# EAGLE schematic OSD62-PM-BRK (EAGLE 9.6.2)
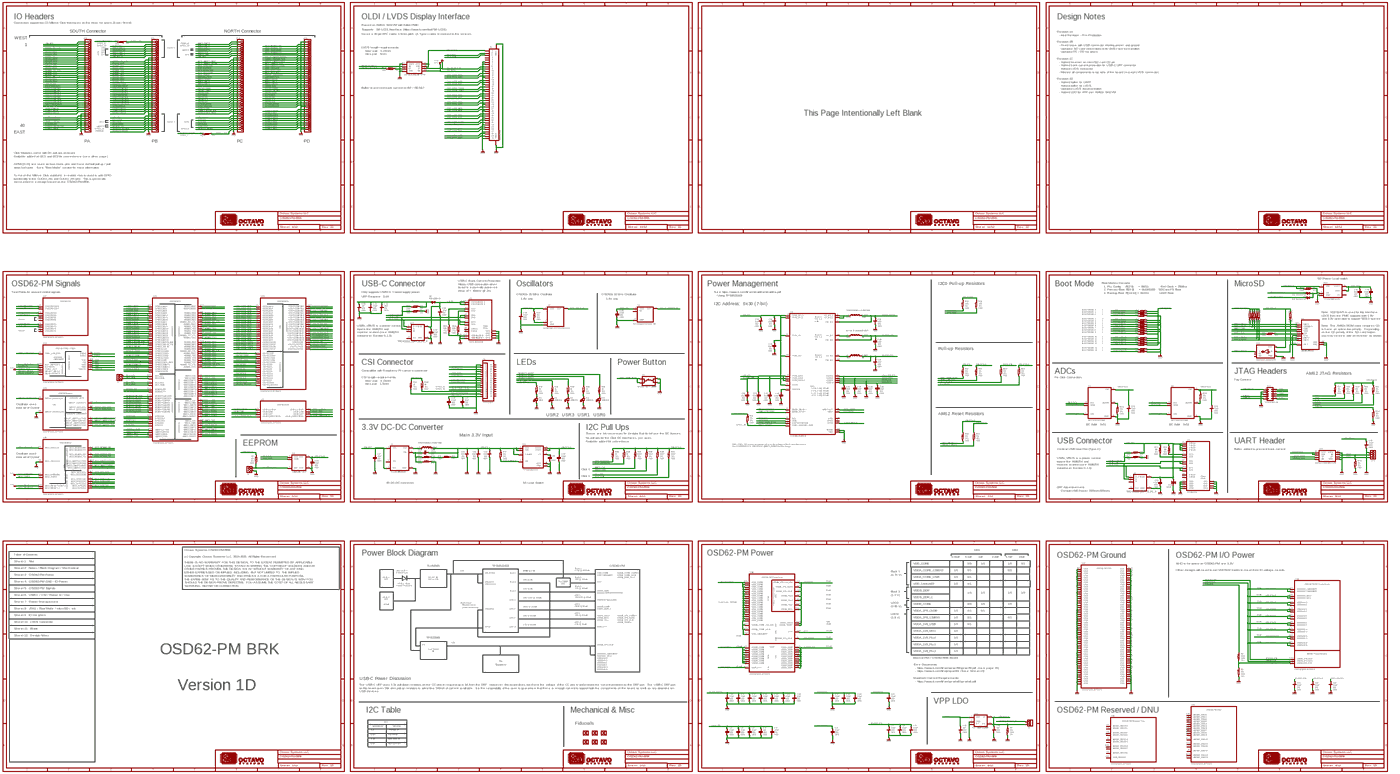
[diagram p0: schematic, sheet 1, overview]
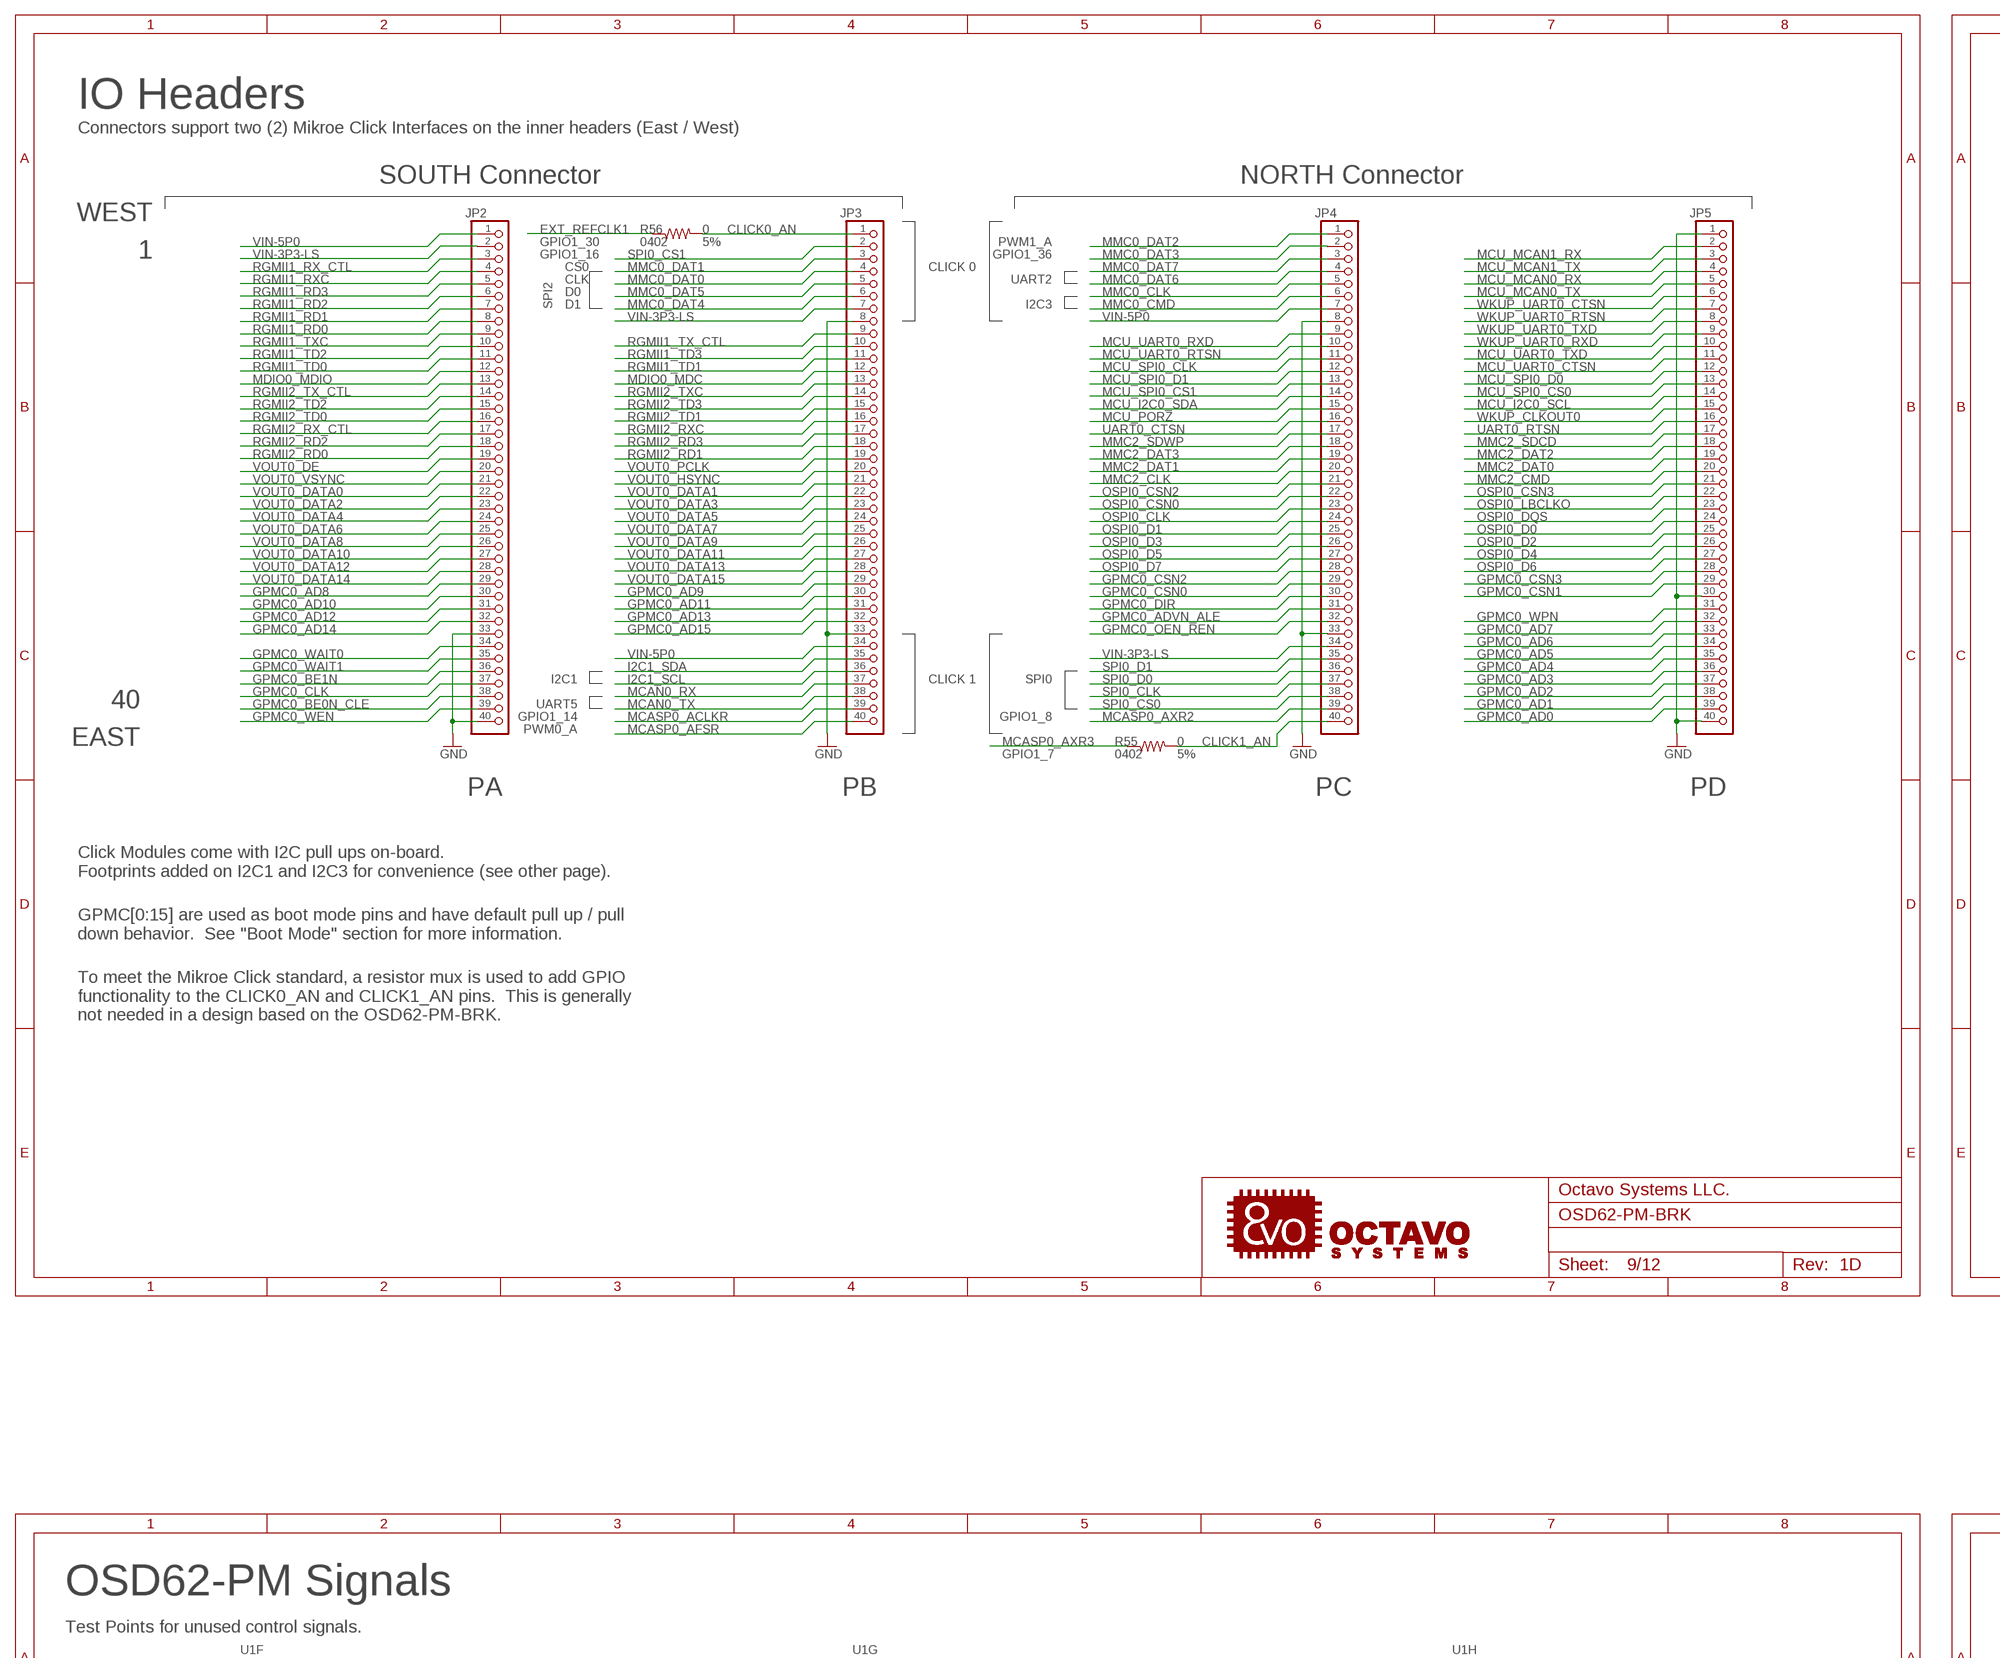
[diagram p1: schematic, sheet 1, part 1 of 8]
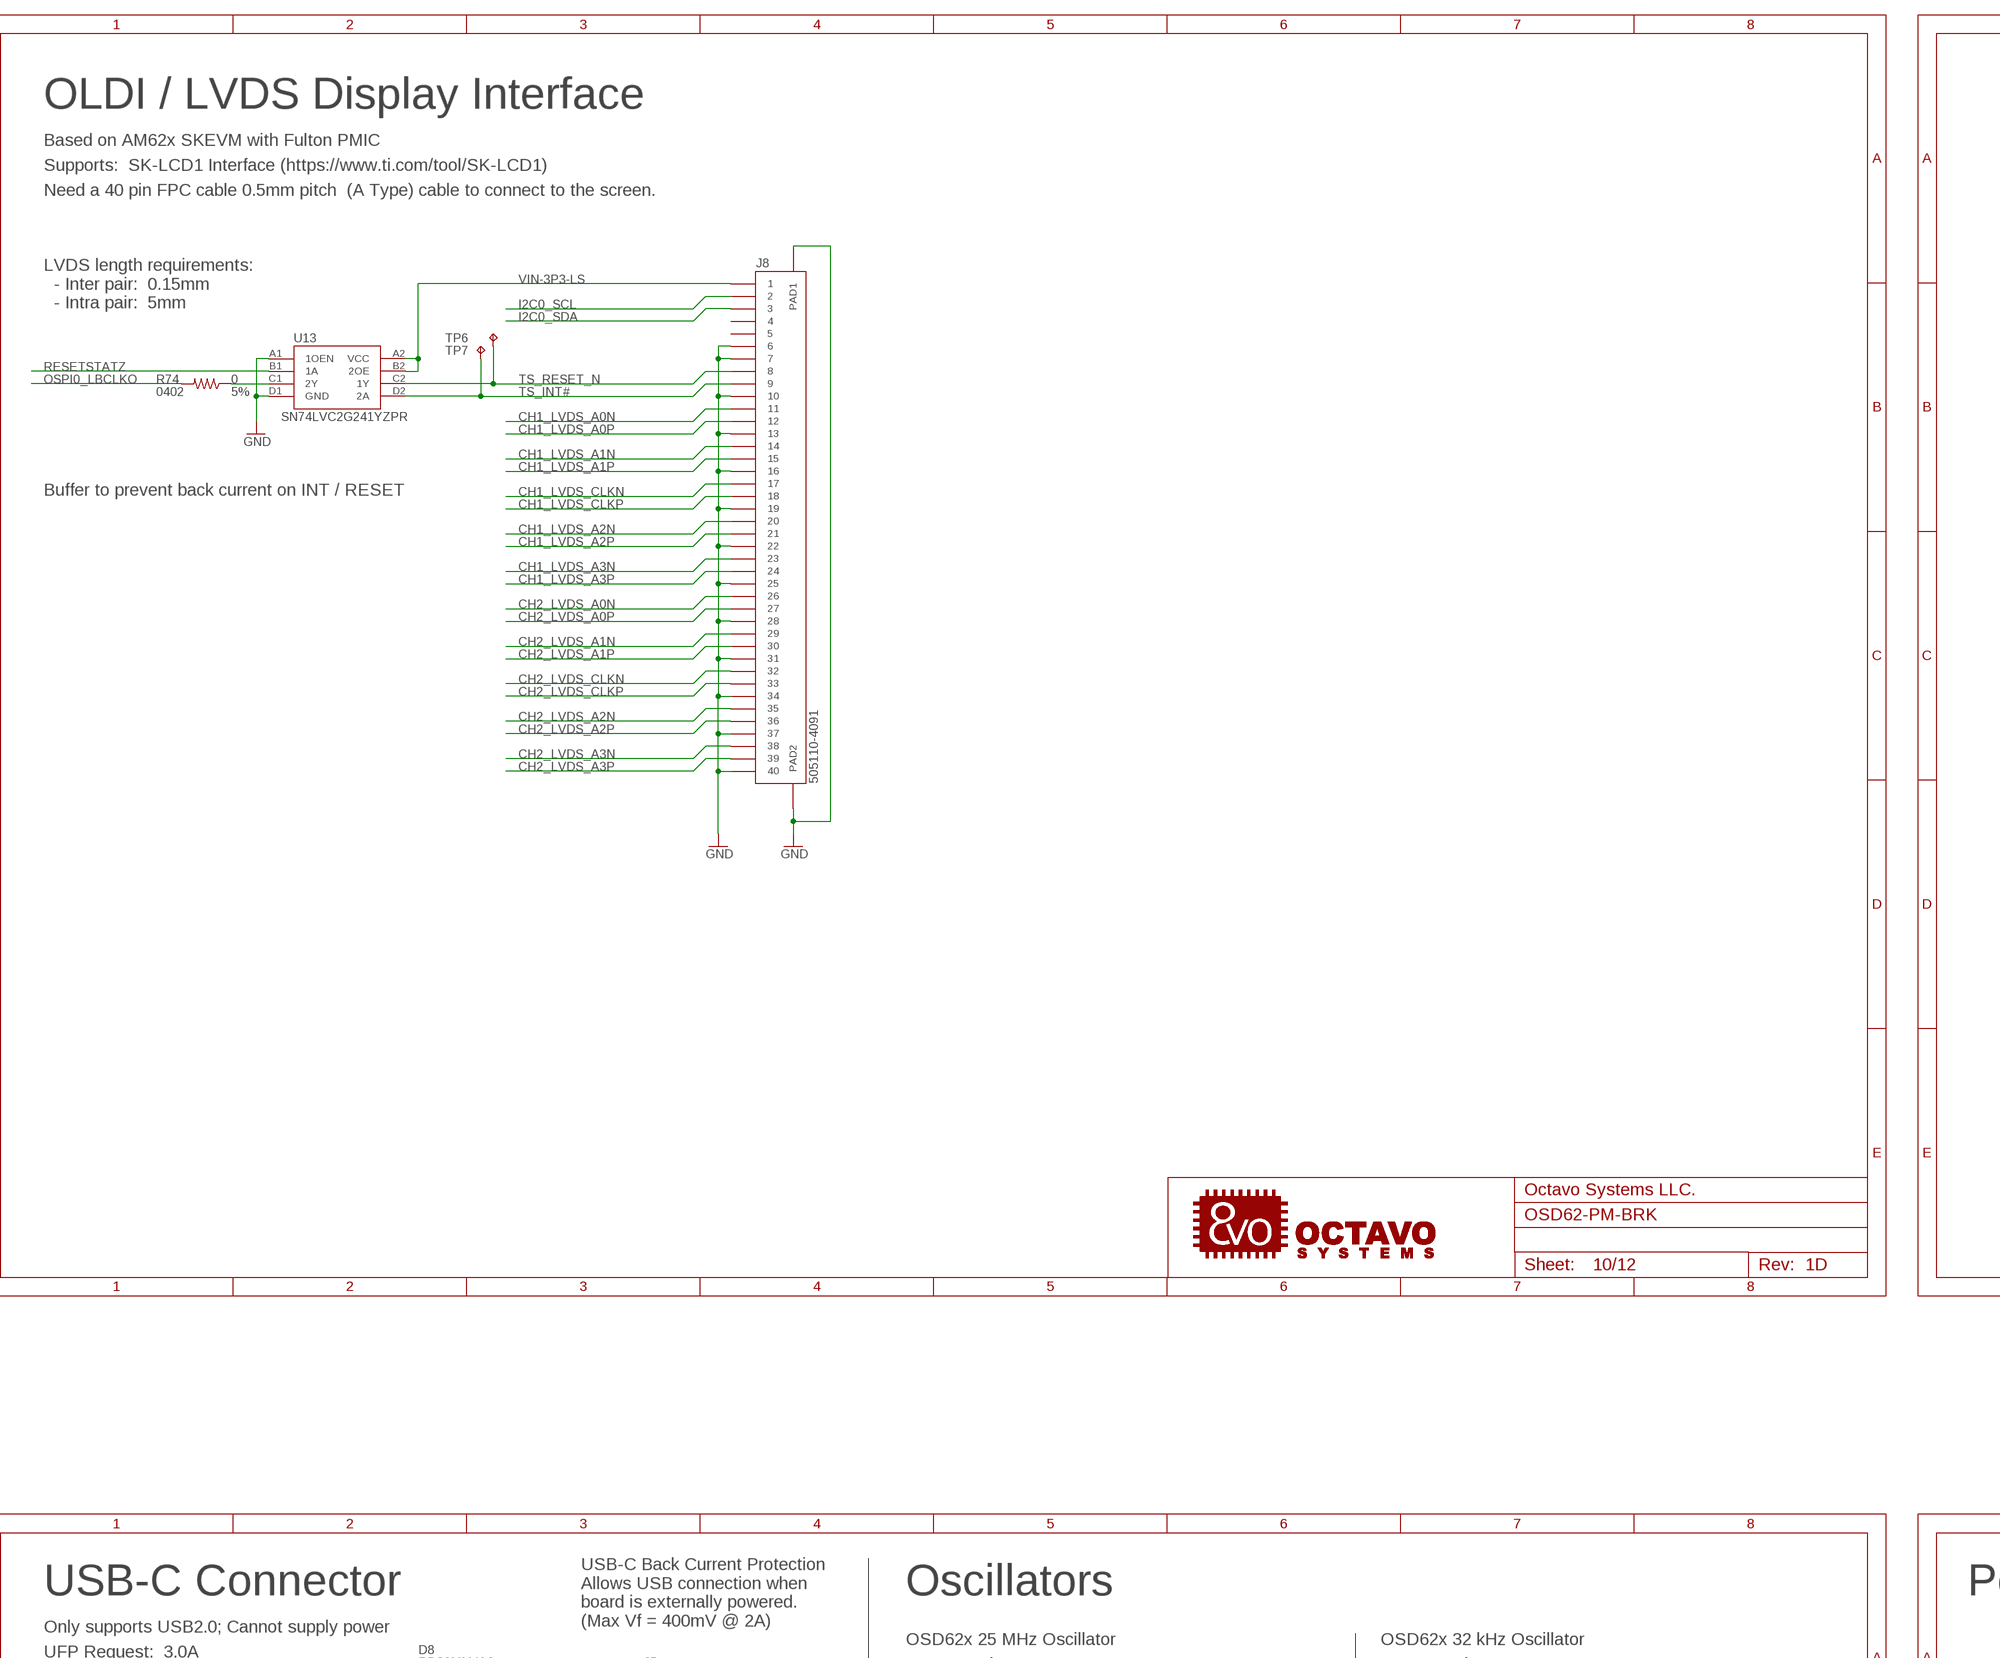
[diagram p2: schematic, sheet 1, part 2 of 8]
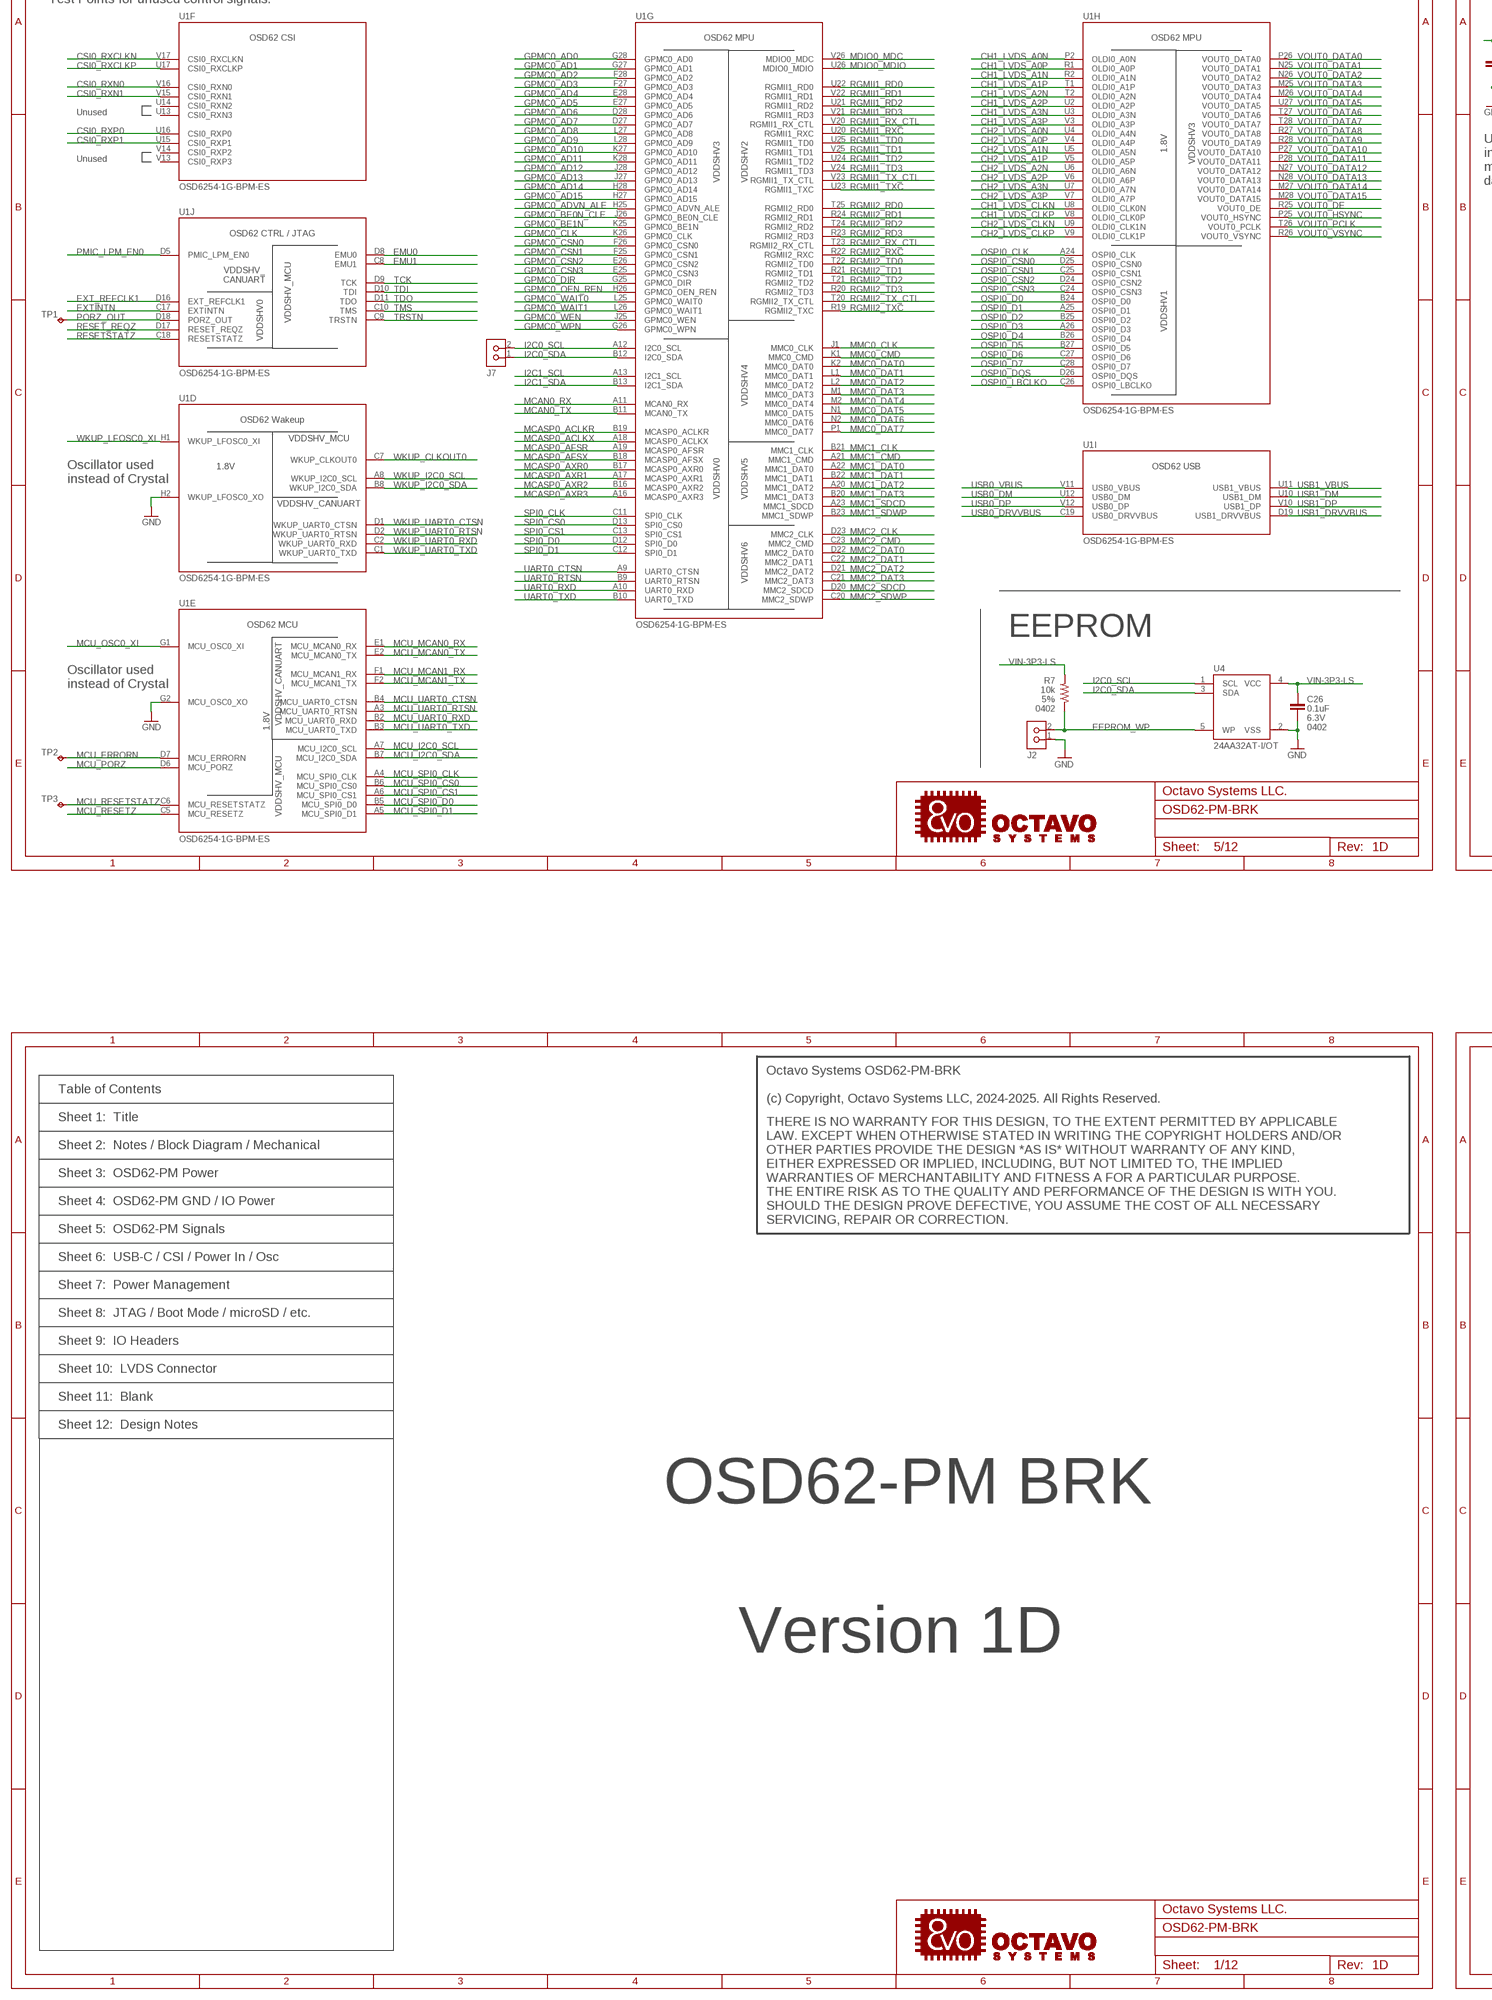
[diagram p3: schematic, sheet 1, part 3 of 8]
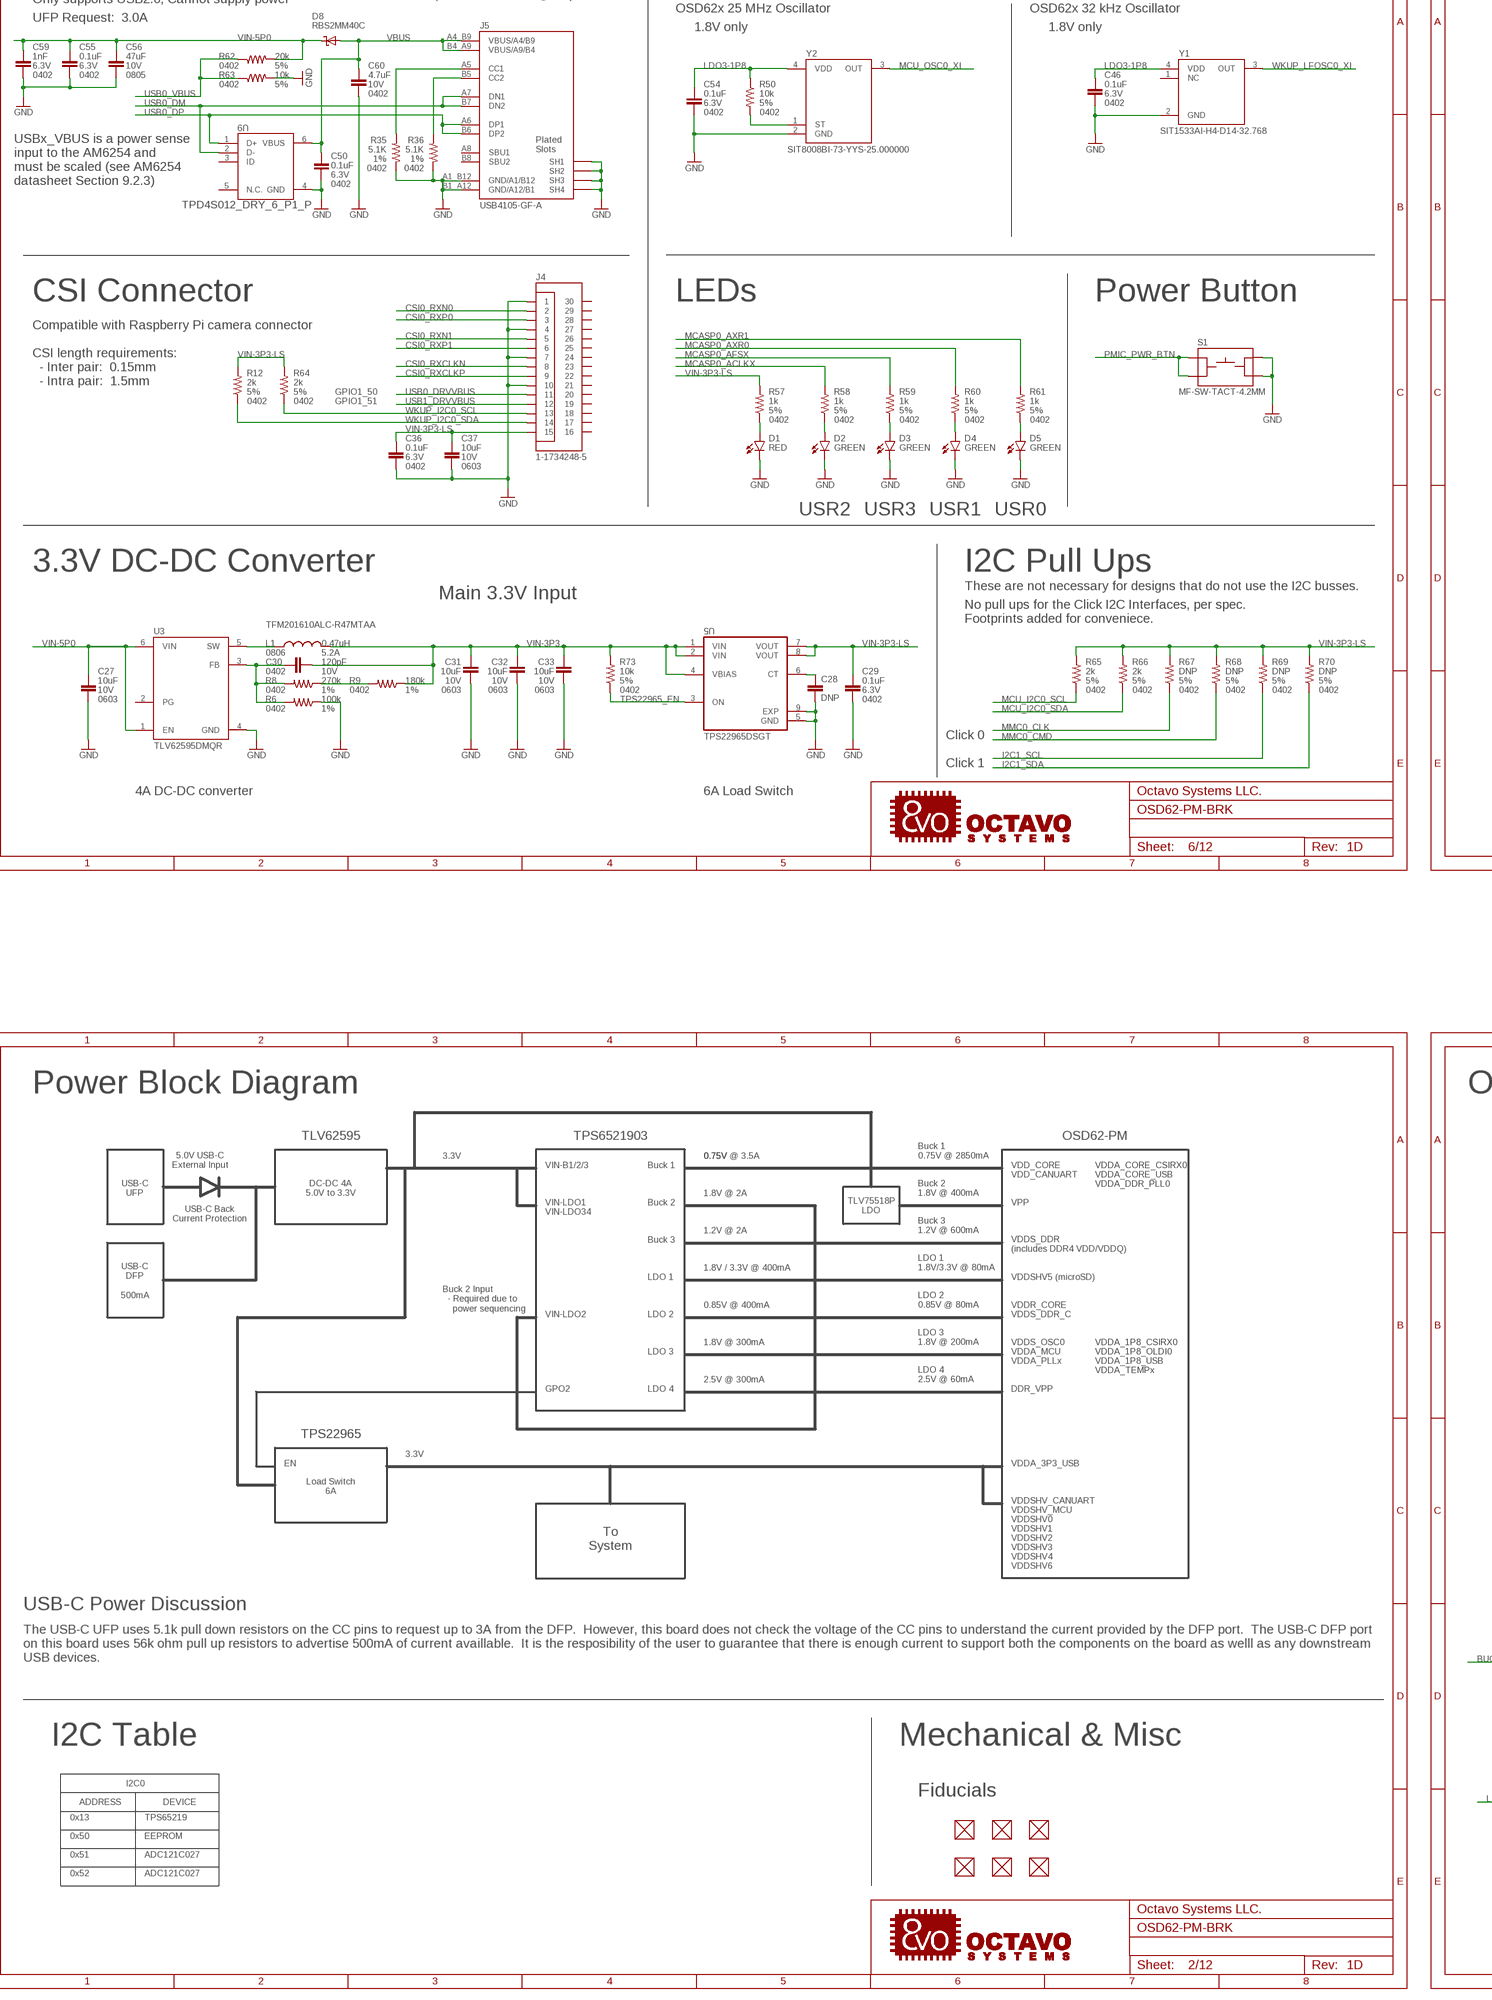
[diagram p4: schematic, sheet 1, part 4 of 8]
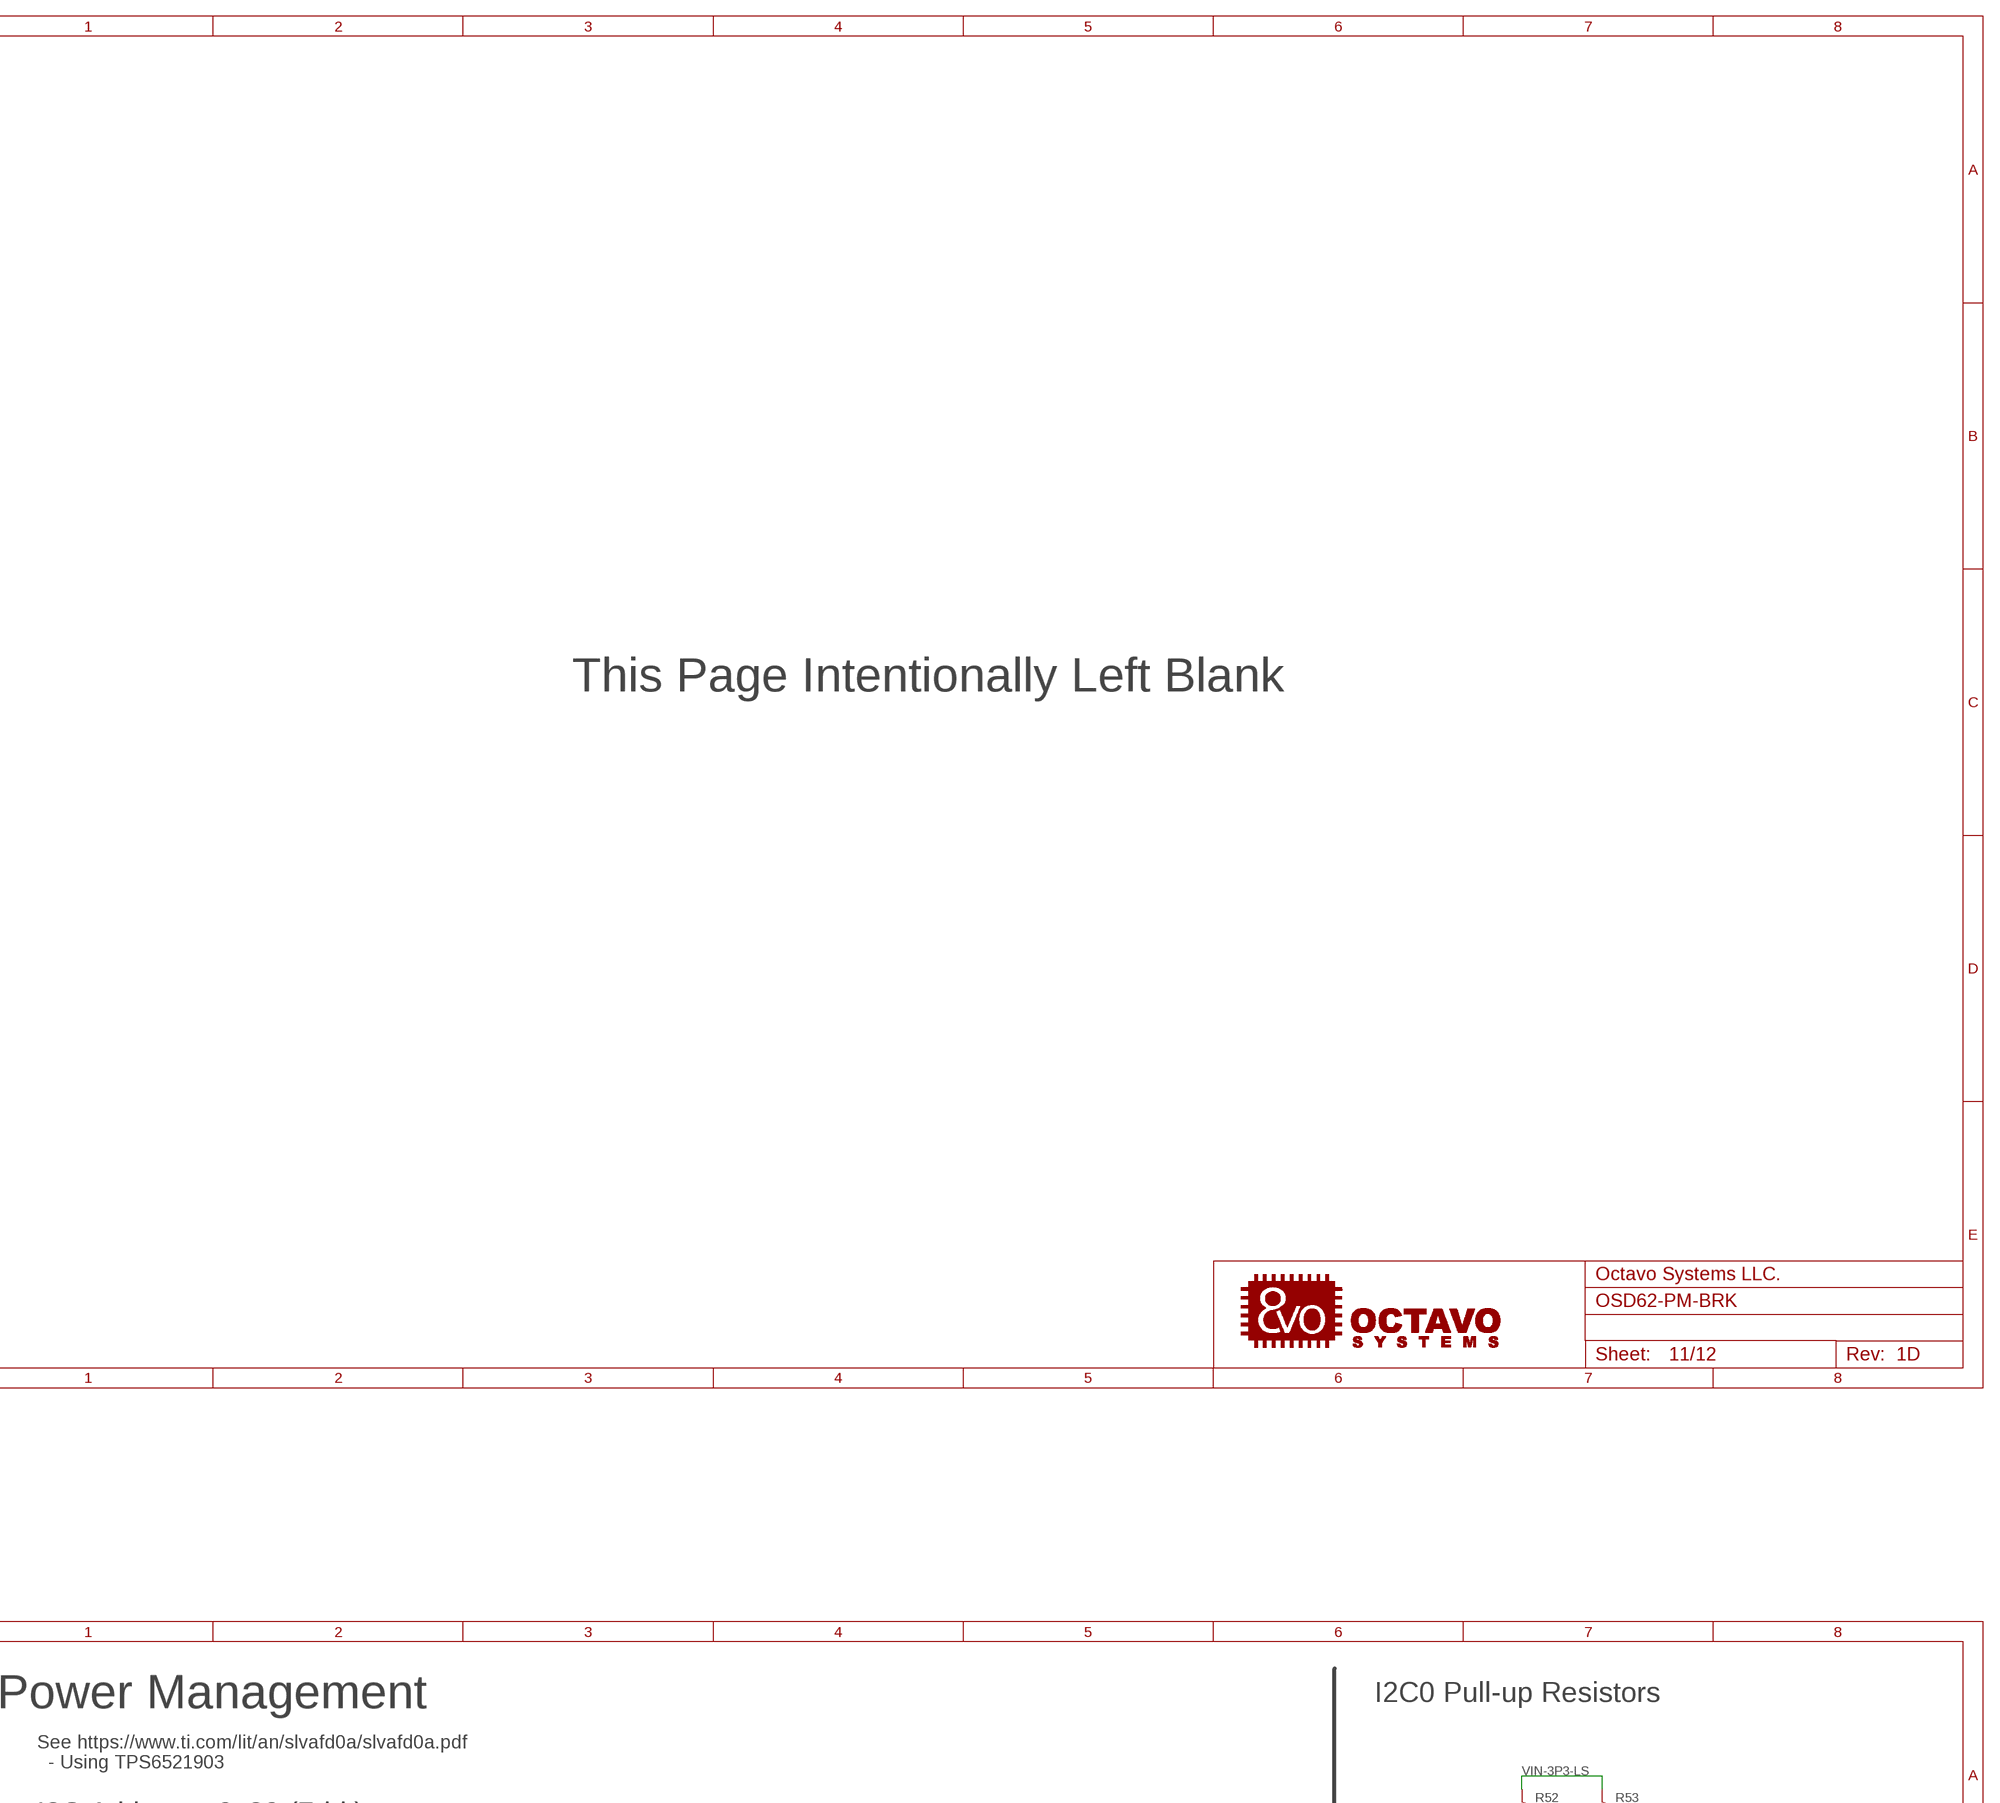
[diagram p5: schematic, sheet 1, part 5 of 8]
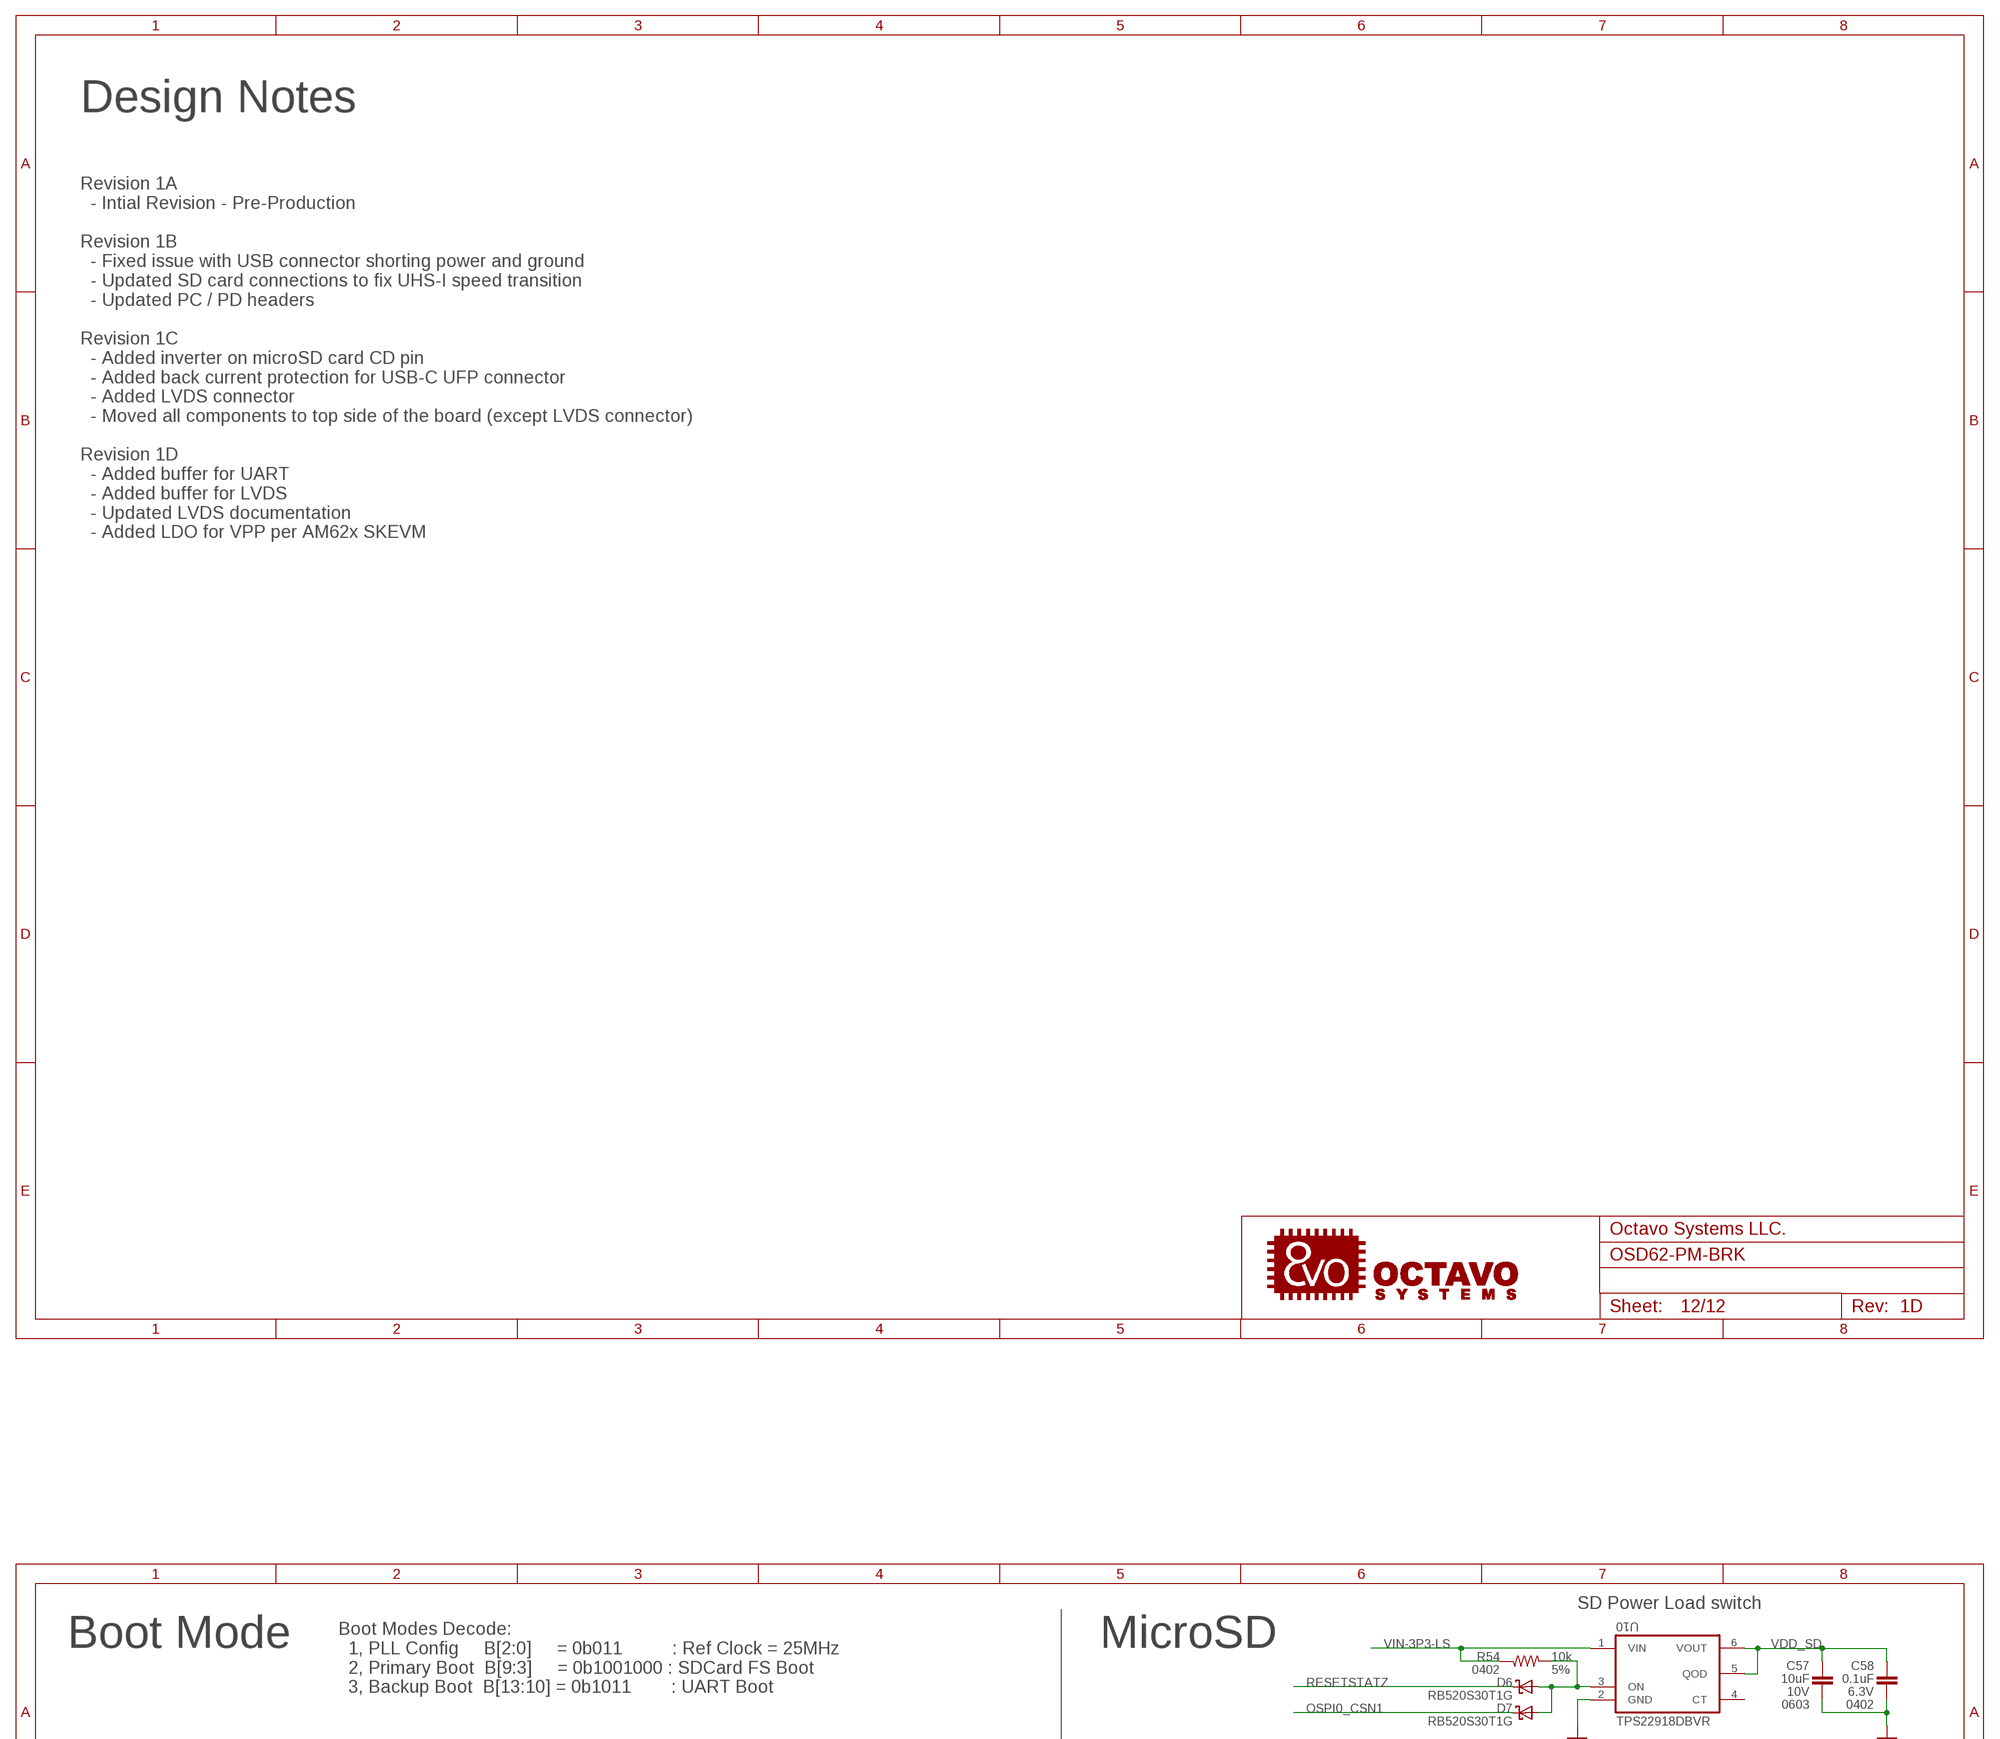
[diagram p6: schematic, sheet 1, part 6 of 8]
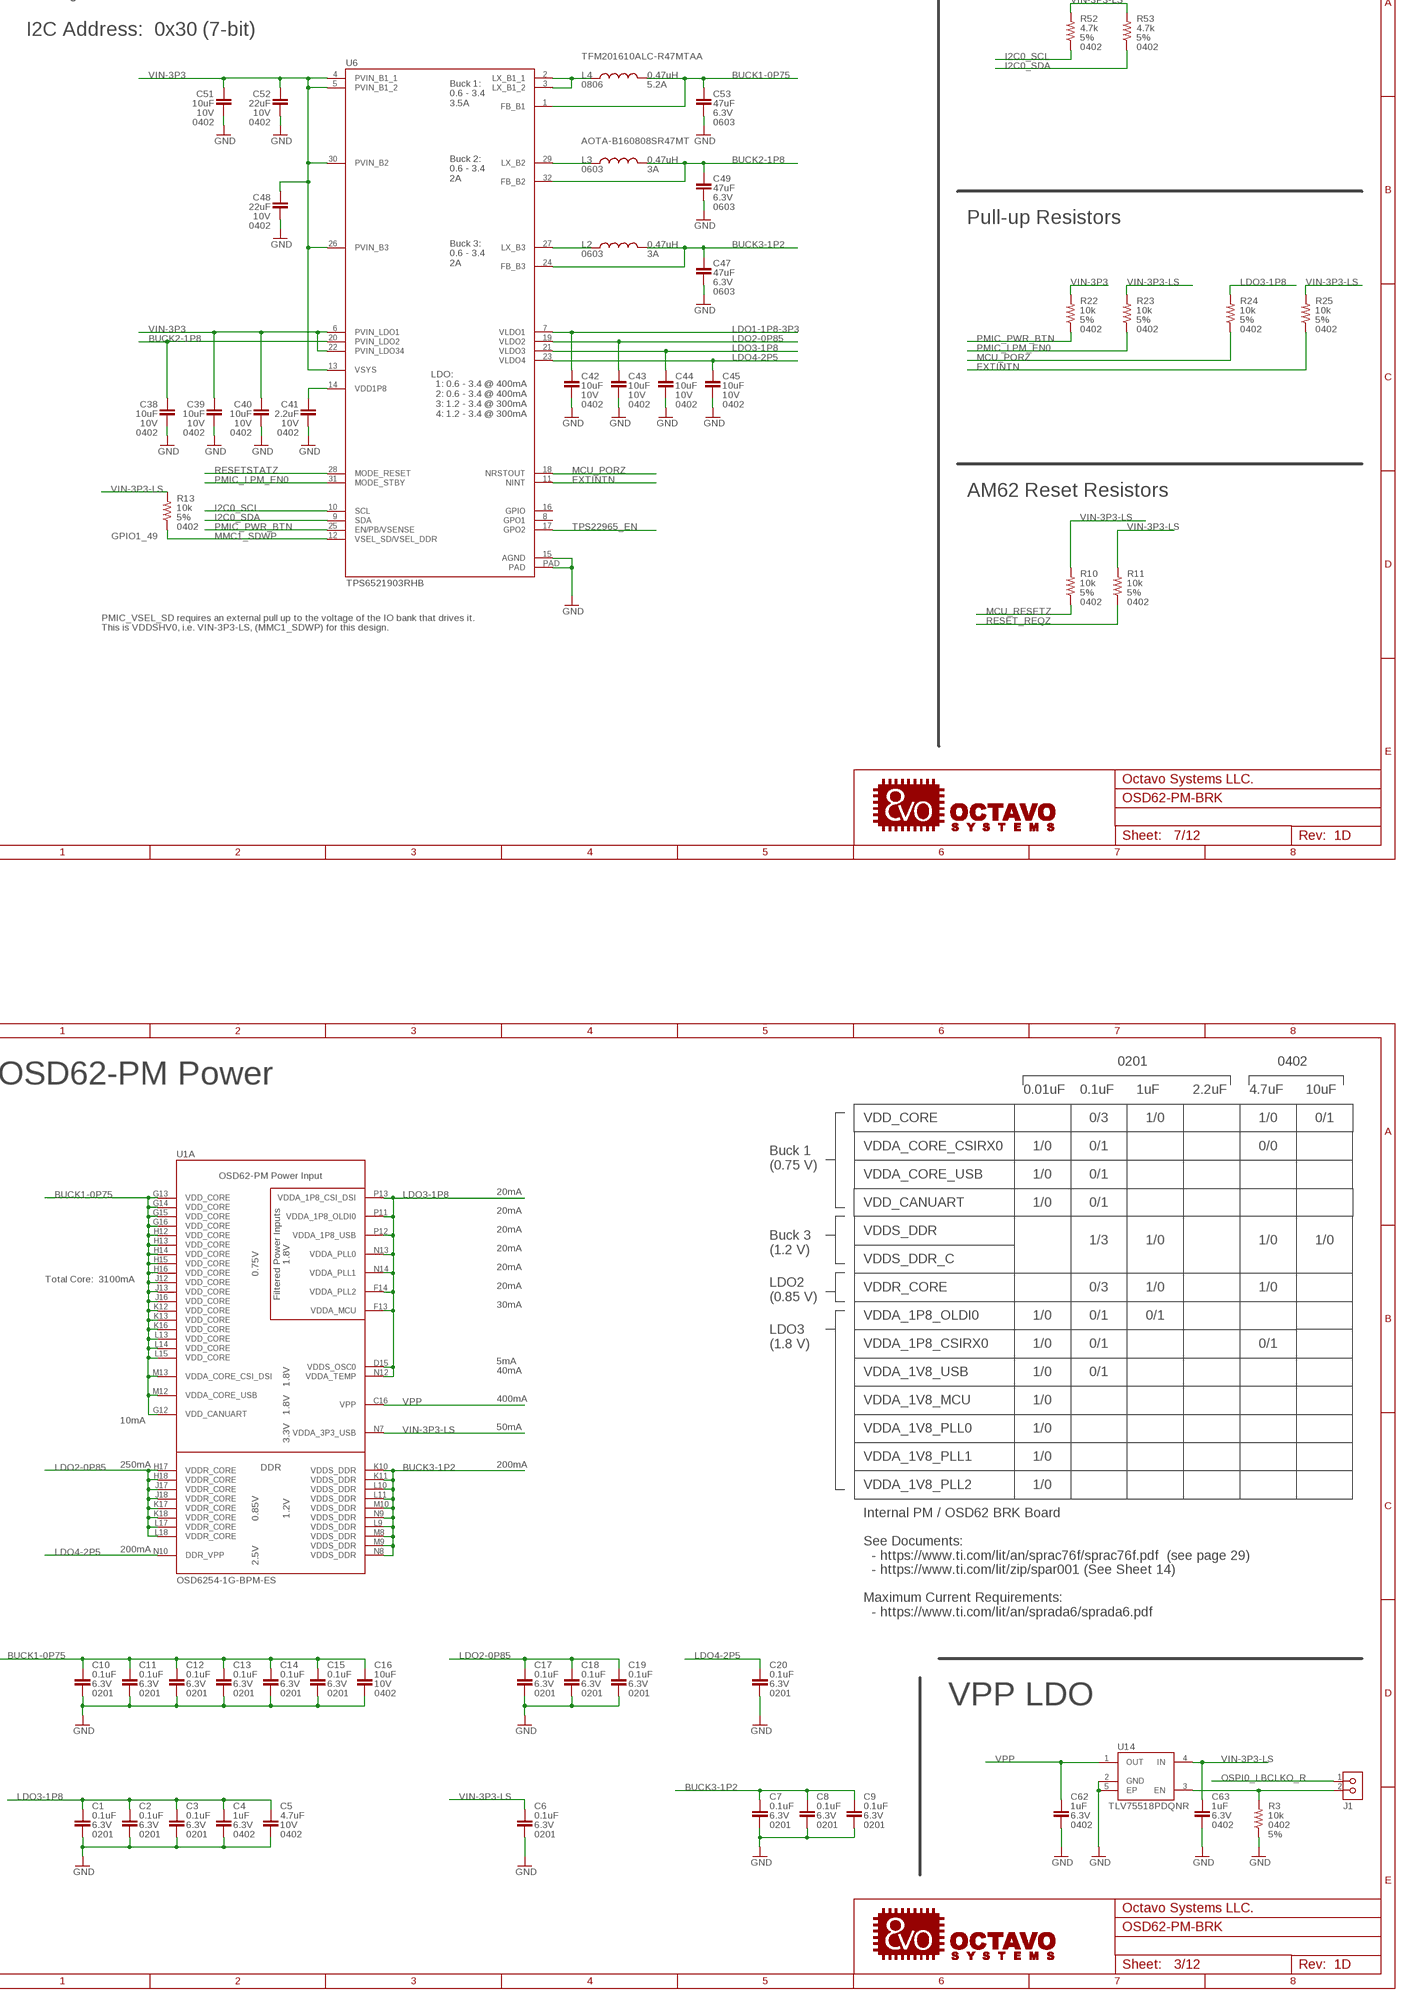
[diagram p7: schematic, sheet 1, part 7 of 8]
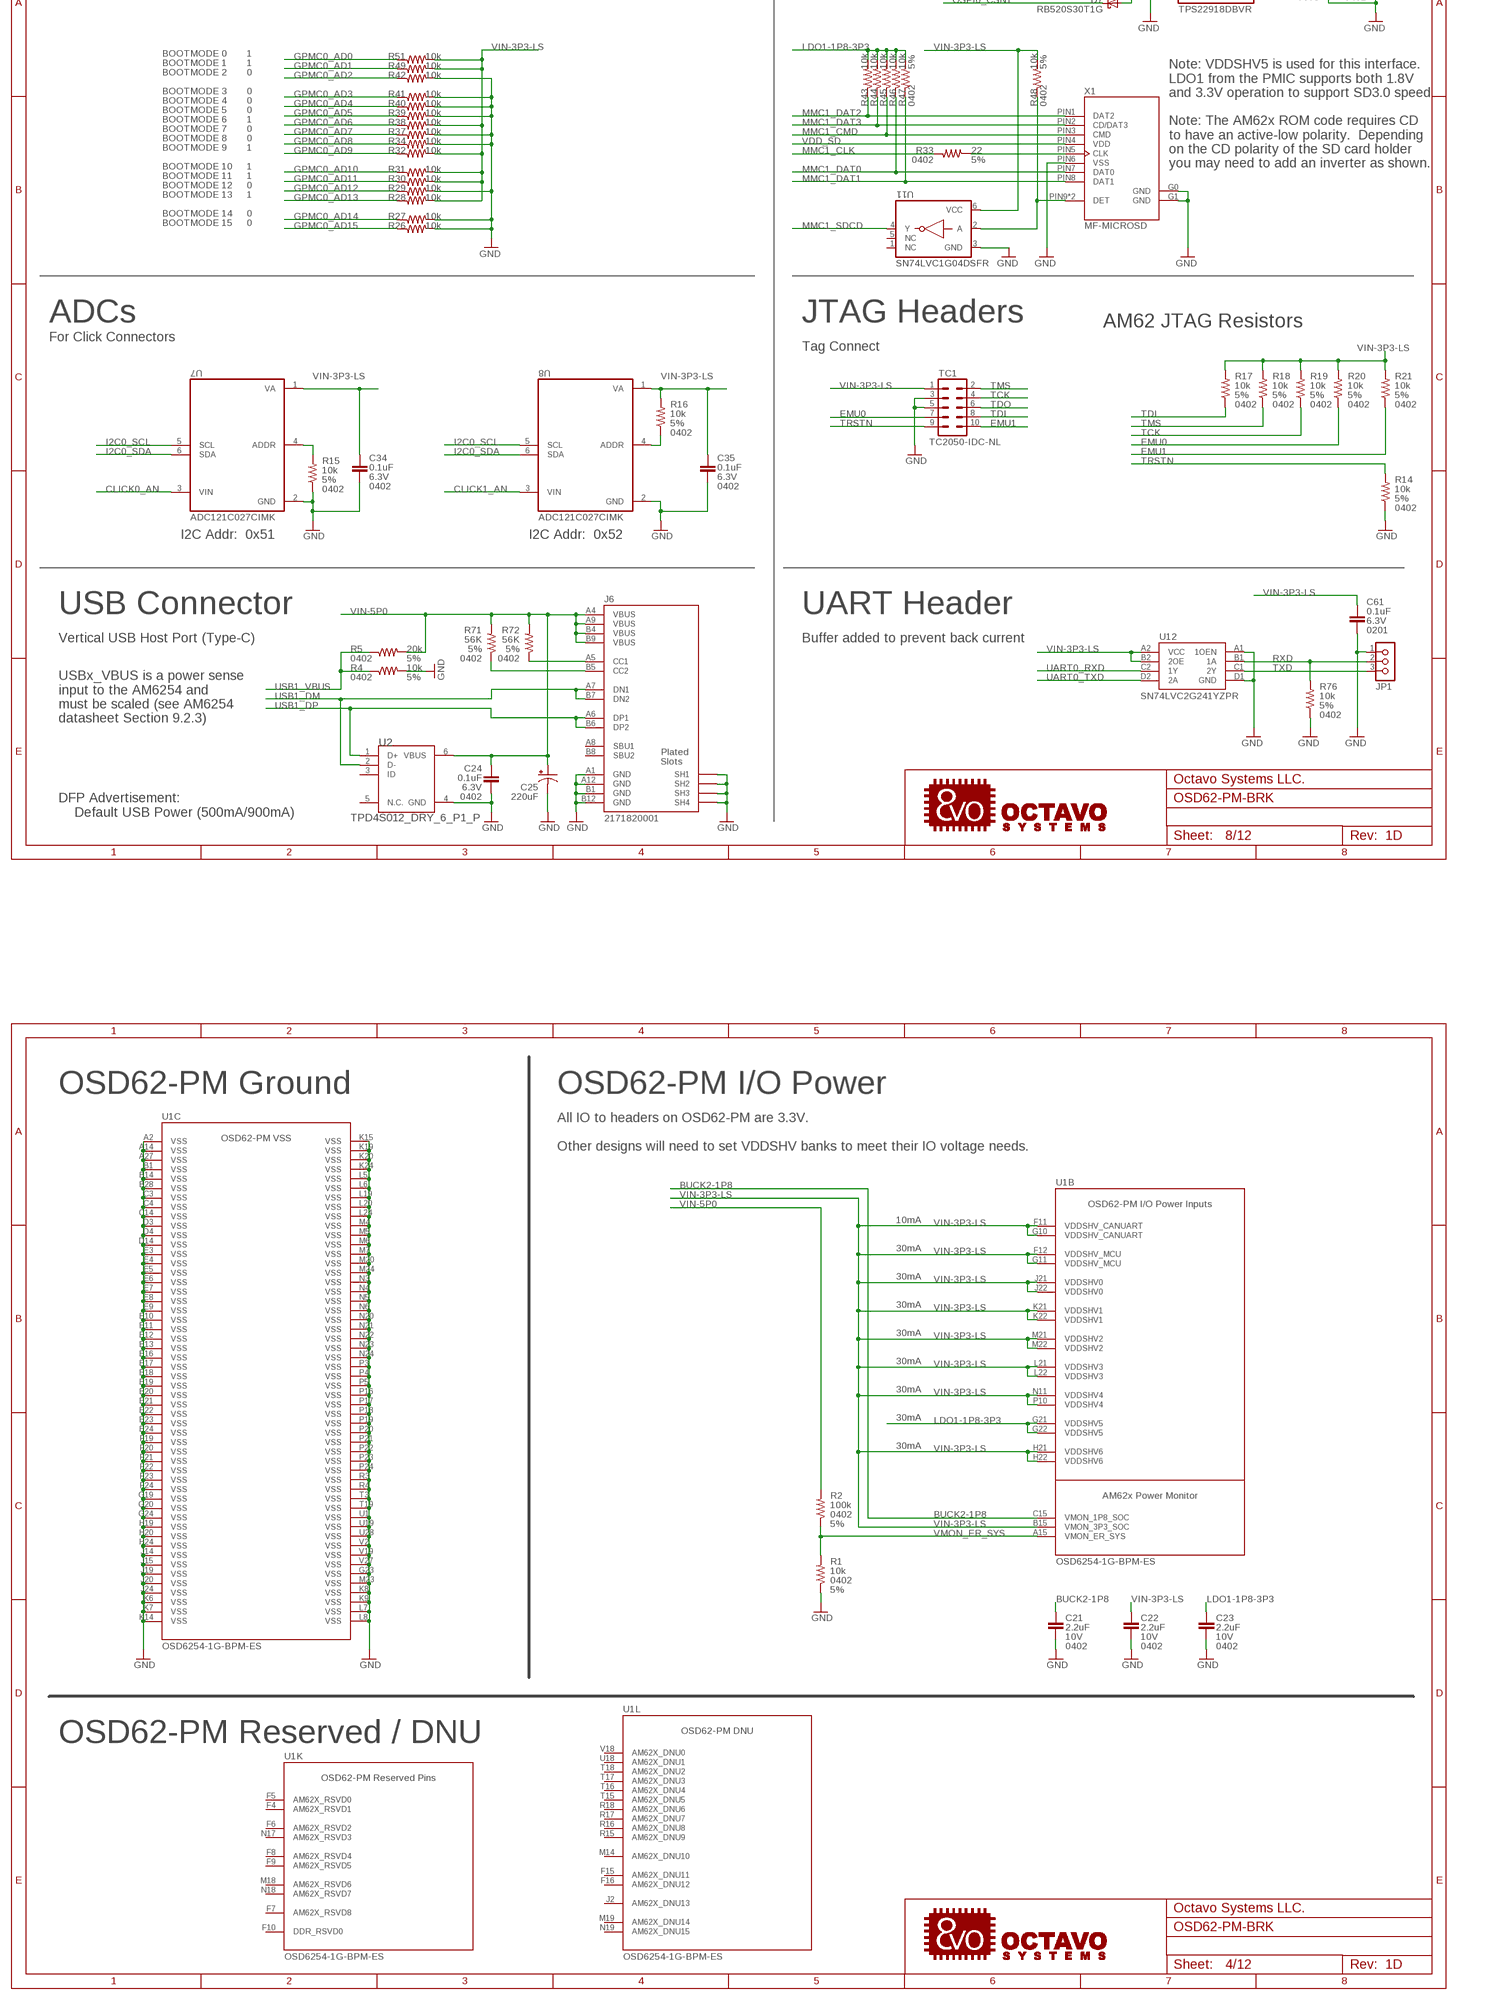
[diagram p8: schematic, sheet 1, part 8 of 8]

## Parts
C1  0.1uF  CC0201  [C0201]
C2  0.1uF  CC0201  [C0201]
C3  0.1uF  CC0201  [C0201]
C4  1uF  CC0402  [C0402]
C5  4.7uF  CC0402  [C0402]
C6  0.1uF  CC0201  [C0201]
C7  0.1uF  CC0201  [C0201]
C8  0.1uF  CC0201  [C0201]
C9  0.1uF  CC0201  [C0201]
C10  0.1uF  CC0201  [C0201]
C11  0.1uF  CC0201  [C0201]
C12  0.1uF  CC0201  [C0201]
C13  0.1uF  CC0201  [C0201]
C14  0.1uF  CC0201  [C0201]
C15  0.1uF  CC0201  [C0201]
C16  10uF  CC0402  [C0402]
C17  0.1uF  CC0201  [C0201]
C18  0.1uF  CC0201  [C0201]
C19  0.1uF  CC0201  [C0201]
C20  0.1uF  CC0201  [C0201]
C21  2.2uF  CC0402  [C0402]
C22  2.2uF  CC0402  [C0402]
C23  2.2uF  CC0402  [C0402]
C24  0.1uF  CC0402  [C0402]
C25  220uF  CPOL-USB/3528-21R  [B/3528-21R]
C26  0.1uF  CC0402  [C0402]
C27  10uF  CC0603  [C0603]
C28  DNP  CC0402  [C0402]
C29  0.1uF  CC0402  [C0402]
C30  120pF  CC0402  [C0402]
C31  10uF  CC0603  [C0603]
C32  10uF  CC0603  [C0603]
C33  10uF  CC0603  [C0603]
C34  0.1uF  CC0402  [C0402]
C35  0.1uF  CC0402  [C0402]
C36  0.1uF  CC0402  [C0402]
C37  10uF  CC0603  [C0603]
C38  10uF  CC0402  [C0402]
C39  10uF  CC0402  [C0402]
C40  10uF  CC0402  [C0402]
C41  2.2uF  CC0402  [C0402]
C42  10uF  CC0402  [C0402]
C43  10uF  CC0402  [C0402]
C44  10uF  CC0402  [C0402]
C45  10uF  CC0402  [C0402]
C46  0.1uF  CC0402  [C0402]
C47  47uF  CC0603  [C0603]
C48  22uF  CC0402  [C0402]
C49  47uF  CC0603  [C0603]
C50  0.1uF  CC0402  [C0402]
C51  10uF  CC0402  [C0402]
C52  22uF  CC0402  [C0402]
C53  47uF  CC0603  [C0603]
C54  0.1uF  CC0402  [C0402]
C55  0.1uF  CC0402  [C0402]
C56  47uF  CC0805  [C0805]
C57  10uF  CC0603  [C0603]
C58  0.1uF  CC0402  [C0402]
C59  1nF  CC0402  [C0402]
C60  4.7uF  CC0402  [C0402]
C61  0.1uF  CC0201  [C0201]
C62  1uF  CC0402  [C0402]
C63  1uF  CC0402  [C0402]
D1  RED  LTST-C191TBKTLALED_EIA-STD  [EIA-STD]
D2  GREEN  LTST-C191TBKTLALED_EIA-STD  [EIA-STD]
D3  GREEN  LTST-C191TBKTLALED_EIA-STD  [EIA-STD]
D4  GREEN  LTST-C191TBKTLALED_EIA-STD  [EIA-STD]
D5  GREEN  LTST-C191TBKTLALED_EIA-STD  [EIA-STD]
D6  RB520S30T1G  [RB520S30T1G]
D7  RB520S30T1G  [RB520S30T1G]
D8  RBS2MM40C  [SOD-123FL]
FUD1  FIDUCIAL  [FIDUCIAL_40MIL]
FUD2  FIDUCIAL  [FIDUCIAL_40MIL]
FUD3  FIDUCIAL  [FIDUCIAL_40MIL]
FUD4  FIDUCIAL  [FIDUCIAL_40MIL]
FUD5  FIDUCIAL  [FIDUCIAL_40MIL]
FUD6  FIDUCIAL  [FIDUCIAL_40MIL]
J1  PINHD-1X21.27  [H1X2-1.27]
J2  PINHD-1X2  [H1X2-2.54]
J4  1-1734248-5  [TE_1-1734248-5]
J5  USB4105-GF-A  [GCT_USB4105-GF-A]
J6  2171820001  [MOLEX_2171820001]
J7  PINHD-1X2  [H1X2-2.54]
J8  505110-4091  [MOLEX_505110-4091]
JP1  PINHD-1X3  [H1X3-2.54]
JP2  PINHD-1X40  [H1X40-2.54]
JP3  PINHD-1X40  [H1X40-2.54]
JP4  PINHD-1X40  [H1X40-2.54]
JP5  PINHD-1X40  [H1X40-2.54]
L1  0.47uH  L0806  [L0806]
L2  0.47uH  L0603  [L0603]
L3  0.47uH  L0603  [L0603]
L4  0.47uH  L0806  [L0806]
R1  10k  R-US_R0402  [R0402]
R2  100k  R-US_R0402  [R0402]
R3  10k  R-US_R0402  [R0402]
R4  10k  R-US_R0402  [R0402]
R5  20k  R-US_R0402  [R0402]
R6  100k  R-US_R0402  [R0402]
R7  10k  R-US_R0402  [R0402]
R8  270k  R-US_R0402  [R0402]
R9  180k  R-US_R0402  [R0402]
R10  10k  R-US_R0402  [R0402]
R11  10k  R-US_R0402  [R0402]
R12  2k  R-US_R0402  [R0402]
R13  10k  R-US_R0402  [R0402]
R14  10k  R-US_R0402  [R0402]
R15  10k  R-US_R0402  [R0402]
R16  10k  R-US_R0402  [R0402]
R17  10k  R-US_R0402  [R0402]
R18  10k  R-US_R0402  [R0402]
R19  10k  R-US_R0402  [R0402]
R20  10k  R-US_R0402  [R0402]
R21  10k  R-US_R0402  [R0402]
R22  10k  R-US_R0402  [R0402]
R23  10k  R-US_R0402  [R0402]
R24  10k  R-US_R0402  [R0402]
R25  10k  R-US_R0402  [R0402]
R26  10k  R-US_R0402  [R0402]
R27  10k  R-US_R0402  [R0402]
R28  10k  R-US_R0402  [R0402]
R29  10k  R-US_R0402  [R0402]
R30  10k  R-US_R0402  [R0402]
R31  10k  R-US_R0402  [R0402]
R32  10k  R-US_R0402  [R0402]
R33  22  R-US_R0402  [R0402]
R34  10k  R-US_R0402  [R0402]
R35  5.1K  R-US_R0402  [R0402]
R36  5.1K  R-US_R0402  [R0402]
R37  10k  R-US_R0402  [R0402]
R38  10k  R-US_R0402  [R0402]
R39  10k  R-US_R0402  [R0402]
R40  10k  R-US_R0402  [R0402]
R41  10k  R-US_R0402  [R0402]
R42  10k  R-US_R0402  [R0402]
R43  10k  R-US_R0402  [R0402]
R44  10k  R-US_R0402  [R0402]
R45  10k  R-US_R0402  [R0402]
R46  10k  R-US_R0402  [R0402]
R47  10k  R-US_R0402  [R0402]
R48  10k  R-US_R0402  [R0402]
R49  10k  R-US_R0402  [R0402]
R50  10k  R-US_R0402  [R0402]
R51  10k  R-US_R0402  [R0402]
R52  4.7k  R-US_R0402  [R0402]
R53  4.7k  R-US_R0402  [R0402]
R54  10k  R-US_R0402  [R0402]
R55  0  R-US_R0402  [R0402]
R56  0  R-US_R0402  [R0402]
R57  1k  R-US_R0402  [R0402]
R58  1k  R-US_R0402  [R0402]
R59  1k  R-US_R0402  [R0402]
R60  1k  R-US_R0402  [R0402]
R61  1k  R-US_R0402  [R0402]
R62  20k  R-US_R0402  [R0402]
R63  10k  R-US_R0402  [R0402]
R64  2k  R-US_R0402  [R0402]
R65  2k  R-US_R0402  [R0402]
R66  2k  R-US_R0402  [R0402]
R67  DNP  R-US_R0402  [R0402]
R68  DNP  R-US_R0402  [R0402]
R69  DNP  R-US_R0402  [R0402]
R70  DNP  R-US_R0402  [R0402]
R71  56K  R-US_R0402  [R0402]
R72  56K  R-US_R0402  [R0402]
R73  10k  R-US_R0402  [R0402]
R74  0  R-US_R0402  [R0402]
R76  10k  R-US_R0402  [R0402]
S1  MF-SW-TACT-4.2MM  TACT_4.2MM  [TACT4.2MM]
TC1  TC2050-IDC-NL  [TC2050-IDC-NL]
TP1  TPB0,65  [TP_B0,65]
TP2  TPB0,65  [TP_B0,65]
TP3  TPB0,65  [TP_B0,65]
TP6  TPB0,65  [TP_B0,65]
TP7  TPB0,65  [TP_B0,65]
U1  OSD6254-1G-BPM-ES  [BGA-500-9X14MM]
U2  TPD4S012_DRY_6_P1_P  [DRY6]
U3  TLV62595DMQR  [DMQ0006A]
U4  24AA32AT-I/OT  [SOT95P280X145-5N]
U5  TPS22965DSGT  [SON50P200X200X80-9N]
U6  TPS6521903RHB  TPS65219-5X5  [RHB0032W]
U7  ADC121C027CIMK  [SOT95P280X110-6N]
U8  ADC121C027CIMK  [SOT95P280X110-6N]
U9  TPD4S012_DRY_6_P1_P  [DRY6]
U10  TPS22918DBVR  [SOT95P280X145-6N]
U11  SN74LVC1G04DSFR  [SON35P100X100X40-6N]
U12  SN74LVC2G241YZPR  [YZP0008]
U13  SN74LVC2G241YZPR  [YZP0008]
U14  TLV75518PDQNR  [DQN0004A]
X1  MF-MICROSD  SD_CARD_SLOT_MICRO_RIGHT  [MF-MICROSD]
Y1  SIT1533AI-H4-D14-32.768  [SIT1533AI_2X1.2MM]
Y2  SIT8008BI-73-YYS-25.000000  [QFN-4-2X1.6MM]

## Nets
3V3_FB: C30.1 R6.2 R8.2 U3.3(FB)
3V3_FB_0: R8.1 R9.2
3V3_SW: L1.1 U3.5(SW)
ADC0_ADDR: R15.2 U7.4(ADDR)
ADC1_ADDR: R16.1 U8.4(ADDR)
BUCK1-0P75: C10.1 C11.1 C12.1 C13.1 C14.1 C15.1 C16.1 C53.1 L4.2 U1.G12(A:VDD_CANUART) U1.G13(A:VDD_CORE) U1.G14(A:VDD_CORE) U1.G15(A:VDD_CORE) U1.G16(A:VDD_CORE) U1.H12(A:VDD_CORE) U1.H13(A:VDD_CORE) U1.H14(A:VDD_CORE) U1.H15(A:VDD_CORE) U1.H16(A:VDD_CORE) U1.J12(A:VDD_CORE) U1.J13(A:VDD_CORE) U1.J16(A:VDD_CORE) U1.K12(A:VDD_CORE) U1.K13(A:VDD_CORE) U1.K16(A:VDD_CORE) U1.L13(A:VDD_CORE) U1.L14(A:VDD_CORE) U1.L15(A:VDD_CORE) U1.M12(A:VDDA_CORE_USB) U1.M13(A:VDDA_CORE_CSI_DSI) U6.1(FB_B1)
BUCK2-1P8: C21.1 C38.1 C49.1 L3.2 U1.C15(B:VMON_1P8_SOC) U6.20(PVIN_LDO2) U6.32(FB_B2)
BUCK3-1P2: C7.1 C8.1 C9.1 C47.1 L2.2 U1.K10(A:VDDS_DDR) U1.K11(A:VDDS_DDR) U1.L9(A:VDDS_DDR) U1.L10(A:VDDS_DDR) U1.L11(A:VDDS_DDR) U1.M8(A:VDDS_DDR) U1.M9(A:VDDS_DDR) U1.M10(A:VDDS_DDR) U1.N8(A:VDDS_DDR) U1.N9(A:VDDS_DDR) U6.24(FB_B3)
CH1_LVDS_A0N: J8.11 U1.P2(H:OLDI0_A0N)
CH1_LVDS_A0P: J8.12 U1.R1(H:OLDI0_A0P)
CH1_LVDS_A1N: J8.14 U1.R2(H:OLDI0_A1N)
CH1_LVDS_A1P: J8.15 U1.T1(H:OLDI0_A1P)
CH1_LVDS_A2N: J8.20 U1.T2(H:OLDI0_A2N)
CH1_LVDS_A2P: J8.21 U1.U2(H:OLDI0_A2P)
CH1_LVDS_A3N: J8.23 U1.U3(H:OLDI0_A3N)
CH1_LVDS_A3P: J8.24 U1.V3(H:OLDI0_A3P)
CH1_LVDS_CLKN: J8.17 U1.U8(H:OLDI0_CLK0N)
CH1_LVDS_CLKP: J8.18 U1.V8(H:OLDI0_CLK0P)
CH2_LVDS_A0N: J8.26 U1.U4(H:OLDI0_A4N)
CH2_LVDS_A0P: J8.27 U1.V4(H:OLDI0_A4P)
CH2_LVDS_A1N: J8.29 U1.U5(H:OLDI0_A5N)
CH2_LVDS_A1P: J8.30 U1.V5(H:OLDI0_A5P)
CH2_LVDS_A2N: J8.35 U1.U6(H:OLDI0_A6N)
CH2_LVDS_A2P: J8.36 U1.V6(H:OLDI0_A6P)
CH2_LVDS_A3N: J8.38 U1.U7(H:OLDI0_A7N)
CH2_LVDS_A3P: J8.39 U1.V7(H:OLDI0_A7P)
CH2_LVDS_CLKN: J8.32 U1.U9(H:OLDI0_CLK1N)
CH2_LVDS_CLKP: J8.33 U1.V9(H:OLDI0_CLK1P)
CLICK0_AN: JP3.1 R56.2 U7.3(VIN)
CLICK1_AN: JP4.40 R55.2 U8.3(VIN)
CSI0_RXCLKN: J4.8 U1.V17(F:CSI0_RXCLKN)
CSI0_RXCLKP: J4.9 U1.U17(F:CSI0_RXCLKP)
CSI0_RXN0: J4.2 U1.V16(F:CSI0_RXN0)
CSI0_RXN1: J4.5 U1.V15(F:CSI0_RXN1)
CSI0_RXP0: J4.3 U1.U16(F:CSI0_RXP0)
CSI0_RXP1: J4.6 U1.U15(F:CSI0_RXP1)
EEPROM_WP: J2.2 R7.1 U4.5(WP)
EMU0: R20.1 TC1.7 U1.D8(J:EMU0)
EMU1: R21.1 TC1.10 U1.C8(J:EMU1)
EXT_REFCLK1: R56.1 U1.D16(J:EXT_REFCLK1)
EXTINTN: R25.1 U1.C17(J:EXTINTN) U6.11(NINT)
GND: C1.2 C2.2 C3.2 C4.2 C5.2 C6.2 C7.2 C8.2 C9.2 C10.2 C11.2 C12.2 C13.2 C14.2 C15.2 C16.2 C17.2 C18.2 C19.2 C20.2 C21.2 C22.2 C23.2 C24.2 C25.- C26.2 C27.2 C28.2 C29.2 C31.2 C32.2 C33.2 C34.2 C35.2 C36.2 C37.2 C38.2 C39.2 C40.2 C41.2 C42.2 C43.2 C44.2 C45.2 C46.2 C47.2 C48.2 C49.2 C50.2 C51.2 C52.2 C53.2 C54.2 C55.2 C56.2 C57.2 C58.2 C59.2 C60.2 C61.2 C62.2 C63.2 D1.2(C) D2.2(C) D3.2(C) D4.2(C) D5.2(C) J2.1 J4.1 J4.4 J4.7 J4.10 J5.A1_B12(GND/A1/B12) J5.B1_A12(GND/A12/B1) J5.SH1_B(SH1) J5.SH1_T(SH1) J5.SH2_B(SH2) J5.SH2_T(SH2) J5.SH3_B(SH3) J5.SH3_T(SH3) J5.SH4_B(SH4) J5.SH4_T(SH4) J6.A1(GND) J6.A12(GND) J6.B1(GND) J6.B12(GND) J6.SH_B_1(SH1) J6.SH_B_2(SH2) J6.SH_B_3(SH3) J6.SH_B_4(SH4) J6.SH_T_1(SH1) J6.SH_T_2(SH2) J6.SH_T_3(SH3) J6.SH_T_4(SH4) J8.6 J8.7 J8.10 J8.13 J8.16 J8.19 J8.22 J8.25 J8.28 J8.31 J8.34 J8.37 J8.40 J8.S1(PAD1) J8.S2(PAD2) JP1.1 JP2.33 JP2.40 JP3.8 JP3.33 JP4.8 JP4.33 JP5.1 JP5.30 JP5.40 R1.1 R3.1 R4.2 R6.1 R14.1 R15.1 R26.2 R27.2 R29.2 R34.2 R35.1 R36.1 R37.2 R39.2 R40.2 R41.2 R42.2 R63.2 R76.1 S1.P$3 S1.P$4 TC1.3 TC1.5 U1.A2(C:VSS) U1.A14(C:VSS) U1.A27(C:VSS) U1.B1(C:VSS) U1.B14(C:VSS) U1.B28(C:VSS) U1.C3(C:VSS) U1.C4(C:VSS) U1.C14(C:VSS) U1.D3(C:VSS) U1.D4(C:VSS) U1.D14(C:VSS) U1.E3(C:VSS) U1.E4(C:VSS) U1.E5(C:VSS) U1.E6(C:VSS) U1.E7(C:VSS) U1.E8(C:VSS) U1.E9(C:VSS) U1.E10(C:VSS) U1.E11(C:VSS) U1.E12(C:VSS) U1.E13(C:VSS) U1.E16(C:VSS) U1.E17(C:VSS) U1.E18(C:VSS) U1.E19(C:VSS) U1.E20(C:VSS) U1.E21(C:VSS) U1.E22(C:VSS) U1.E23(C:VSS) U1.E24(C:VSS) U1.F19(C:VSS) U1.F20(C:VSS) U1.F21(C:VSS) U1.F22(C:VSS) U1.F23(C:VSS) U1.F24(C:VSS) U1.G2(E:MCU_OSC0_XO) U1.G19(C:VSS) U1.G20(C:VSS) U1.G23(C:VSS) U1.G24(C:VSS) U1.H2(D:WKUP_LFOSC0_XO) U1.H19(C:VSS) U1.H20(C:VSS) U1.H24(C:VSS) U1.J14(C:VSS) U1.J15(C:VSS) U1.J19(C:VSS) U1.J20(C:VSS) U1.J24(C:VSS) U1.K6(C:VSS) U1.K7(C:VSS) U1.K8(C:VSS) U1.K9(C:VSS) U1.K14(C:VSS) U1.K15(C:VSS) U1.K19(C:VSS) U1.K20(C:VSS) U1.K24(C:VSS) U1.L5(C:VSS) U1.L6(C:VSS) U1.L7(C:VSS) U1.L8(C:VSS) U1.L19(C:VSS) U1.L20(C:VSS) U1.L24(C:VSS) U1.M4(C:VSS) U1.M5(C:VSS) U1.M6(C:VSS) U1.M7(C:VSS) U1.M20(C:VSS) U1.M23(C:VSS) U1.M24(C:VSS) U1.N3(C:VSS) U1.N4(C:VSS) U1.N5(C:VSS) U1.N6(C:VSS) U1.N20(C:VSS) U1.N21(C:VSS) U1.N22(C:VSS) U1.N23(C:VSS) U1.N24(C:VSS) U1.P3(C:VSS) U1.P4(C:VSS) U1.P5(C:VSS) U1.P16(C:VSS) U1.P17(C:VSS) U1.P18(C:VSS) U1.P19(C:VSS) U1.P20(C:VSS) U1.P21(C:VSS) U1.P22(C:VSS) U1.P23(C:VSS) U1.P24(C:VSS) U1.R3(C:VSS) U1.R4(C:VSS) U1.T3(C:VSS) U1.T19(C:VSS) U1.U1(C:VSS) U1.U19(C:VSS) U1.U28(C:VSS) U1.V2(C:VSS) U1.V19(C:VSS) U1.V27(C:VSS) U2.4(GND) U3.4(GND) U4.2(VSS) U5.5(GND) U5.9(EXP) U6.15(AGND) U6.PAD U7.2(GND) U8.2(GND) U9.4(GND) U10.2(GND) U11.3(GND) U12.A1(1OEN) U12.D1(GND) U13.A1(1OEN) U13.D1(GND) U14.2(GND) U14.5(EP) X1.G0(GND) X1.G1(GND) X1.PIN6(VSS) Y1.2(GND) Y2.2(GND)
GPMC0_AD0: JP5.39 R51.1 U1.G28(G:GPMC0_AD0)
GPMC0_AD1: JP5.38 R49.1 U1.G27(G:GPMC0_AD1)
GPMC0_AD2: JP5.37 R42.1 U1.F28(G:GPMC0_AD2)
GPMC0_AD3: JP5.36 R41.1 U1.F27(G:GPMC0_AD3)
GPMC0_AD4: JP5.35 R40.1 U1.E28(G:GPMC0_AD4)
GPMC0_AD5: JP5.34 R39.1 U1.E27(G:GPMC0_AD5)
GPMC0_AD6: JP5.33 R38.1 U1.D28(G:GPMC0_AD6)
GPMC0_AD7: JP5.32 R37.1 U1.D27(G:GPMC0_AD7)
GPMC0_AD8: JP2.29 R34.1 U1.L27(G:GPMC0_AD8)
GPMC0_AD9: JP3.29 R32.1 U1.L28(G:GPMC0_AD9)
GPMC0_AD10: JP2.30 R31.1 U1.K27(G:GPMC0_AD10)
GPMC0_AD11: JP3.30 R30.1 U1.K28(G:GPMC0_AD11)
GPMC0_AD12: JP2.31 R29.1 U1.J28(G:GPMC0_AD12)
GPMC0_AD13: JP3.31 R28.1 U1.J27(G:GPMC0_AD13)
GPMC0_AD14: JP2.32 R27.1 U1.H28(G:GPMC0_AD14)
GPMC0_AD15: JP3.32 R26.1 U1.H27(G:GPMC0_AD15)
GPMC0_ADVN_ALE: JP4.31 U1.H25(G:GPMC0_ADVN_ALE)
GPMC0_BE0N_CLE: JP2.38 U1.J26(G:GPMC0_BE0N_CLE)
GPMC0_BE1N: JP2.36 U1.K25(G:GPMC0_BE1N)
GPMC0_CLK: JP2.37 U1.K26(G:GPMC0_CLK)
GPMC0_CSN0: JP4.29 U1.F26(G:GPMC0_CSN0)
GPMC0_CSN1: JP5.29 U1.F25(G:GPMC0_CSN1)
GPMC0_CSN2: JP4.28 U1.E26(G:GPMC0_CSN2)
GPMC0_CSN3: JP5.28 U1.E25(G:GPMC0_CSN3)
GPMC0_DIR: JP4.30 U1.G25(G:GPMC0_DIR)
GPMC0_OEN_REN: JP4.32 U1.H26(G:GPMC0_OEN_REN)
GPMC0_WAIT0: JP2.34 U1.L25(G:GPMC0_WAIT0)
GPMC0_WAIT1: JP2.35 U1.L26(G:GPMC0_WAIT1)
GPMC0_WEN: JP2.39 U1.J25(G:GPMC0_WEN)
GPMC0_WPN: JP5.31 U1.G26(G:GPMC0_WPN)
I2C0_SCL: J7.2 J8.2 R52.1 U1.A12(G:I2C0_SCL) U4.1(SCL) U6.10(SCL) U7.5(SCL) U8.5(SCL)
I2C0_SDA: J7.1 J8.3 R53.1 U1.B12(G:I2C0_SDA) U4.3(SDA) U6.9(SDA) U7.6(SDA) U8.6(SDA)
I2C1_SCL: JP3.36 R69.1 U1.A13(G:I2C1_SCL)
I2C1_SDA: JP3.35 R70.1 U1.B13(G:I2C1_SDA)
LDO1-1P8-3P3: C23.1 C42.1 R43.2 R44.2 R45.2 R46.2 R47.2 U1.G21(B:VDDSHV5) U1.G22(B:VDDSHV5) U6.7(VLDO1)
LDO2-0P85: C17.1 C18.1 C19.1 C43.1 U1.H17(A:VDDR_CORE) U1.H18(A:VDDR_CORE) U1.J17(A:VDDR_CORE) U1.J18(A:VDDR_CORE) U1.K17(A:VDDR_CORE) U1.K18(A:VDDR_CORE) U1.L17(A:VDDR_CORE) U1.L18(A:VDDR_CORE) U6.19(VLDO2)
LDO3-1P8: C1.1 C2.1 C3.1 C4.1 C5.1 C44.1 C46.1 C54.1 R24.2 R50.1 U1.D15(A:VDDS_OSC0) U1.F13(A:VDDA_MCU) U1.F14(A:VDDA_PLL2) U1.N12(A:VDDA_TEMP) U1.N13(A:VDDA_PLL0) U1.N14(A:VDDA_PLL1) U1.P11(A:VDDA_1P8_OLDI0) U1.P12(A:VDDA_1P8_USB) U1.P13(A:VDDA_1P8_CSI_DSI) U6.21(VLDO3) Y1.4(VDD) Y2.4(VDD)
LDO4-2P5: C20.1 C45.1 U1.N10(A:DDR_VPP) U6.23(VLDO4)
LED1: D1.1(A) R57.1
LED2: D2.1(A) R58.1
LED3: D3.1(A) R59.1
LED4: D4.1(A) R60.1
LED5: D5.1(A) R61.1
LX_B1: L4.1 U6.2(LX_B1_1) U6.3(LX_B1_2)
LX_B2: L3.1 U6.29(LX_B2)
LX_B3: L2.1 U6.27(LX_B3)
MCAN0_RX: JP3.37 U1.A11(G:MCAN0_RX)
MCAN0_TX: JP3.38 U1.B11(G:MCAN0_TX)
MCASP0_ACLKR: JP3.39 U1.B19(G:MCASP0_ACLKR)
MCASP0_ACLKX: R58.2 U1.A18(G:MCASP0_ACLKX)
MCASP0_AFSR: JP3.40 U1.A19(G:MCASP0_AFSR)
MCASP0_AFSX: R59.2 U1.B18(G:MCASP0_AFSX)
MCASP0_AXR0: R60.2 U1.B17(G:MCASP0_AXR0)
MCASP0_AXR1: R61.2 U1.A17(G:MCASP0_AXR1)
MCASP0_AXR2: JP4.39 U1.B16(G:MCASP0_AXR2)
MCASP0_AXR3: R55.1 U1.A16(G:MCASP0_AXR3)
MCU_ERRORN: TP2.TP U1.D7(E:MCU_ERRORN)
MCU_I2C0_SCL: JP5.14 R65.1 U1.A7(E:MCU_I2C0_SCL)
MCU_I2C0_SDA: JP4.14 R66.1 U1.B7(E:MCU_I2C0_SDA)
MCU_MCAN0_RX: JP5.4 U1.E1(E:MCU_MCAN0_RX)
MCU_MCAN0_TX: JP5.5 U1.E2(E:MCU_MCAN0_TX)
MCU_MCAN1_RX: JP5.2 U1.F1(E:MCU_MCAN1_RX)
MCU_MCAN1_TX: JP5.3 U1.F2(E:MCU_MCAN1_TX)
MCU_OSC0_XI: U1.G1(E:MCU_OSC0_XI) Y2.3(OUT)
MCU_PORZ: JP4.15 R24.1 U1.D6(E:MCU_PORZ) U6.18(NRSTOUT)
MCU_RESETSTATZ: TP3.TP U1.C6(E:MCU_RESETSTATZ)
MCU_RESETZ: R10.1 U1.C5(E:MCU_RESETZ)
MCU_SPI0_CLK: JP4.11 U1.A4(E:MCU_SPI0_CLK)
MCU_SPI0_CS0: JP5.13 U1.B6(E:MCU_SPI0_CS0)
MCU_SPI0_CS1: JP4.13 U1.A6(E:MCU_SPI0_CS1)
MCU_SPI0_D0: JP5.12 U1.B5(E:MCU_SPI0_D0)
MCU_SPI0_D1: JP4.12 U1.A5(E:MCU_SPI0_D1)
MCU_UART0_CTSN: JP5.11 U1.B4(E:MCU_UART0_CTSN)
MCU_UART0_RTSN: JP4.10 U1.A3(E:MCU_UART0_RTSN)
MCU_UART0_RXD: JP4.9 U1.B2(E:MCU_UART0_RXD)
MCU_UART0_TXD: JP5.10 U1.B3(E:MCU_UART0_TXD)
MDIO0_MDC: JP3.12 U1.V26(G:MDIO0_MDC)
MDIO0_MDIO: JP2.12 U1.U26(G:MDIO0_MDIO)
MMC0_CLK: JP4.5 R67.1 U1.J1(G:MMC0_CLK)
MMC0_CMD: JP4.6 R68.1 U1.K1(G:MMC0_CMD)
MMC0_DAT0: JP3.4 U1.K2(G:MMC0_DAT0)
MMC0_DAT1: JP3.3 U1.L1(G:MMC0_DAT1)
MMC0_DAT2: JP4.1 U1.L2(G:MMC0_DAT2)
MMC0_DAT3: JP4.2 U1.M1(G:MMC0_DAT3)
MMC0_DAT4: JP3.6 U1.M2(G:MMC0_DAT4)
MMC0_DAT5: JP3.5 U1.N1(G:MMC0_DAT5)
MMC0_DAT6: JP4.4 U1.N2(G:MMC0_DAT6)
MMC0_DAT7: JP4.3 U1.P1(G:MMC0_DAT7)
MMC1_CLK: R33.2 U1.B21(G:MMC1_CLK)
MMC1_CLK_R: R33.1 X1.PIN5(CLK)
MMC1_CMD: R45.1 U1.A21(G:MMC1_CMD) X1.PIN3(CMD)
MMC1_DAT0: R46.1 U1.A22(G:MMC1_DAT0) X1.PIN7(DAT0)
MMC1_DAT1: R47.1 U1.B22(G:MMC1_DAT1) X1.PIN8(DAT1)
MMC1_DAT2: R43.1 U1.A20(G:MMC1_DAT2) X1.PIN1(DAT2)
MMC1_DAT3: R44.1 U1.B20(G:MMC1_DAT3) X1.PIN2(CD/DAT3)
MMC1_SDCD: U1.A23(G:MMC1_SDCD) U11.4(Y)
MMC1_SDWP: R13.1 U1.B23(G:MMC1_SDWP) U6.12(VSEL_SD/VSEL_DDR)
MMC2_CLK: JP4.20 U1.D23(G:MMC2_CLK)
MMC2_CMD: JP5.20 U1.C23(G:MMC2_CMD)
MMC2_DAT0: JP5.19 U1.D22(G:MMC2_DAT0)
MMC2_DAT1: JP4.19 U1.C22(G:MMC2_DAT1)
MMC2_DAT2: JP5.18 U1.D21(G:MMC2_DAT2)
MMC2_DAT3: JP4.18 U1.C21(G:MMC2_DAT3)
MMC2_SDCD: JP5.17 U1.D20(G:MMC2_SDCD)
MMC2_SDWP: JP4.17 U1.C20(G:MMC2_SDWP)
MPU_HFOSC_EN: R50.2 Y2.1(ST)
OSPI0_CLK: JP4.23 U1.A24(H:OSPI0_CLK)
OSPI0_CSN0: JP4.22 U1.D25(H:OSPI0_CSN0)
OSPI0_CSN1: D7.CATHODE(C) U1.C25(H:OSPI0_CSN1)
OSPI0_CSN2: JP4.21 U1.D24(H:OSPI0_CSN2)
OSPI0_CSN3: JP5.21 U1.C24(H:OSPI0_CSN3)
OSPI0_D0: JP5.24 U1.B24(H:OSPI0_D0)
OSPI0_D1: JP4.24 U1.A25(H:OSPI0_D1)
OSPI0_D2: JP5.25 U1.B25(H:OSPI0_D2)
OSPI0_D3: JP4.25 U1.A26(H:OSPI0_D3)
OSPI0_D4: JP5.26 U1.B26(H:OSPI0_D4)
OSPI0_D5: JP4.26 U1.B27(H:OSPI0_D5)
OSPI0_D6: JP5.27 U1.C27(H:OSPI0_D6)
OSPI0_D7: JP4.27 U1.C28(H:OSPI0_D7)
OSPI0_DQS: JP5.23 U1.D26(H:OSPI0_DQS)
OSPI0_LBCLKO: JP5.22 R74.2 U1.C26(H:OSPI0_LBCLKO)
OSPI0_LBCLKO_R: J1.1 R74.1 U13.C1(2Y)
PMIC_LPM_EN0: R23.1 U1.D5(J:PMIC_LPM_EN0) U6.31(MODE_STBY)
PMIC_PWR_BTN: R22.1 S1.P$1 S1.P$2 U6.25(EN/PB/VSENSE)
PORZ_OUT: TP1.TP U1.D18(J:PORZ_OUT)
RESET_REQZ: R11.1 U1.D17(J:RESET_REQZ)
RESETSTATZ: D6.CATHODE(C) U1.C18(J:RESETSTATZ) U6.28(MODE_RESET) U13.B1(1A)
RGMII1_RD0: JP2.8 U1.U22(G:RGMII1_RD0)
RGMII1_RD1: JP2.7 U1.V22(G:RGMII1_RD1)
RGMII1_RD2: JP2.6 U1.U21(G:RGMII1_RD2)
RGMII1_RD3: JP2.5 U1.V21(G:RGMII1_RD3)
RGMII1_RX_CTL: JP2.3 U1.V20(G:RGMII1_RX_CTL)
RGMII1_RXC: JP2.4 U1.U20(G:RGMII1_RXC)
RGMII1_TD0: JP2.11 U1.U25(G:RGMII1_TD0)
RGMII1_TD1: JP3.11 U1.V25(G:RGMII1_TD1)
RGMII1_TD2: JP2.10 U1.U24(G:RGMII1_TD2)
RGMII1_TD3: JP3.10 U1.V24(G:RGMII1_TD3)
RGMII1_TX_CTL: JP3.9 U1.V23(G:RGMII1_TX_CTL)
RGMII1_TXC: JP2.9 U1.U23(G:RGMII1_TXC)
RGMII2_RD0: JP2.18 U1.T25(G:RGMII2_RD0)
RGMII2_RD1: JP3.18 U1.R24(G:RGMII2_RD1)
RGMII2_RD2: JP2.17 U1.T24(G:RGMII2_RD2)
RGMII2_RD3: JP3.17 U1.R23(G:RGMII2_RD3)
RGMII2_RX_CTL: JP2.16 U1.T23(G:RGMII2_RX_CTL)
RGMII2_RXC: JP3.16 U1.R22(G:RGMII2_RXC)
RGMII2_TD0: JP2.15 U1.T22(G:RGMII2_TD0)
RGMII2_TD1: JP3.15 U1.R21(G:RGMII2_TD1)
RGMII2_TD2: JP2.14 U1.T21(G:RGMII2_TD2)
RGMII2_TD3: JP3.14 U1.R20(G:RGMII2_TD3)
RGMII2_TX_CTL: JP2.13 U1.T20(G:RGMII2_TX_CTL)
RGMII2_TXC: JP3.13 U1.R19(G:RGMII2_TXC)
RXD: JP1.2 R76.2 U12.B1(1A)
SD_LS_ON: D6.ANODE(A) D7.ANODE(A) R54.2 U10.3(ON)
SDCD_INV: R48.1 U11.2(A) X1.PIN9(DET) X1.PIN10(DET)
SPI0_CLK: JP4.37 U1.C11(G:SPI0_CLK)
SPI0_CS0: JP4.38 U1.D13(G:SPI0_CS0)
SPI0_CS1: JP3.2 U1.C13(G:SPI0_CS1)
SPI0_D0: JP4.36 U1.D12(G:SPI0_D0)
SPI0_D1: JP4.35 U1.C12(G:SPI0_D1)
TCK: R19.1 TC1.4 U1.D9(J:TCK)
TDI: R17.1 TC1.8 U1.D10(J:TDI)
TDO: TC1.6 U1.D11(J:TDO)
TMS: R18.1 TC1.2 U1.C10(J:TMS)
TPS22965_CT: C28.1 U5.6(CT)
TPS22965_EN: R73.1 U5.3(ON) U6.17(GPO2)
TRSTN: R14.2 TC1.9 U1.C9(J:TRSTN)
TS_INT#: J8.9 TP7.TP U13.D2(2A)
TS_RESET_N: J8.8 TP6.TP U13.C2(1Y)
TXD: JP1.3 U12.C1(2Y)
UART0_CTSN: JP4.16 U1.A9(G:UART0_CTSN)
UART0_RTSN: JP5.16 U1.B9(G:UART0_RTSN)
UART0_RXD: U1.A10(G:UART0_RXD) U12.C2(1Y)
UART0_TXD: U1.B10(G:UART0_TXD) U12.D2(2A)
USB0_CC1: J5.A5(CC1) R35.2
USB0_CC2: J5.B5(CC2) R36.2
USB0_DM: J5.A7(DN1) J5.B7(DN2) U1.U12(I:USB0_DM) U9.2(D-)
USB0_DP: J5.A6(DP1) J5.B6(DP2) U1.V12(I:USB0_DP) U9.1(D+)
USB0_DRVVBUS: J4.11 U1.C19(I:USB0_DRVVBUS)
USB0_VBUS: R62.1 R63.1 U1.V11(I:USB0_VBUS)
USB1_CC1: J6.A5(CC1) R72.1
USB1_CC2: J6.B5(CC2) R71.1
USB1_DM: J6.A7(DN1) J6.B7(DN2) U1.U10(I:USB1_DM) U2.2(D-)
USB1_DP: J6.A6(DP1) J6.B6(DP2) U1.V10(I:USB1_DP) U2.1(D+)
USB1_DRVVBUS: J4.12 U1.D19(I:USB1_DRVVBUS)
USB1_VBUS: R4.1 R5.1 U1.U11(I:USB1_VBUS)
VBUS: C50.1 C60.1 D8.A J5.A4_B9(VBUS/A4/B9) J5.B4_A9(VBUS/A9/B4) U9.6(VBUS)
VDD1P8_CAP: C41.1 U6.14(VDD1P8)
VDD_SD: C57.1 C58.1 U10.5(QOD) U10.6(VOUT) X1.PIN4(VDD)
VIN-3P3: C30.2 C31.1 C32.1 C33.1 C39.1 C40.1 C48.1 C51.1 C52.1 L1.2 R9.1 R22.2 R73.2 U5.1(VIN) U5.2(VIN) U5.4(VBIAS) U6.4(PVIN_B1_1) U6.5(PVIN_B1_2) U6.6(PVIN_LDO1) U6.13(VSYS) U6.22(PVIN_LDO34) U6.26(PVIN_B3) U6.30(PVIN_B2)
VIN-3P3-LS: C6.1 C22.1 C26.1 C29.1 C34.1 C35.1 C36.1 C37.1 C61.1 C63.1 J4.15 J8.1 JP2.2 JP3.7 JP4.34 R7.2 R10.2 R11.2 R12.2 R13.2 R16.2 R17.2 R18.2 R19.2 R20.2 R21.2 R23.2 R25.2 R28.2 R30.2 R31.2 R32.2 R38.2 R48.2 R49.2 R51.2 R52.2 R53.2 R54.1 R57.2 R64.2 R65.2 R66.2 R67.2 R68.2 R69.2 R70.2 TC1.1 U1.B15(B:VMON_3P3_SOC) U1.F11(B:VDDSHV_CANUART) U1.F12(B:VDDSHV_MCU) U1.G10(B:VDDSHV_CANUART) U1.G11(B:VDDSHV_MCU) U1.H21(B:VDDSHV6) U1.H22(B:VDDSHV6) U1.J21(B:VDDSHV0) U1.J22(B:VDDSHV0) U1.K21(B:VDDSHV1) U1.K22(B:VDDSHV1) U1.L21(B:VDDSHV3) U1.L22(B:VDDSHV3) U1.M21(B:VDDSHV2) U1.M22(B:VDDSHV2) U1.N7(A:VDDA_3P3_USB) U1.N11(B:VDDSHV4) U1.P10(B:VDDSHV4) U4.4(VCC) U5.7(VOUT) U5.8(VOUT) U7.1(VA) U8.1(VA) U10.1(VIN) U11.6(VCC) U12.A2(VCC) U12.B2(2OE) U13.A2(VCC) U13.B2(2OE) U14.4(IN)
VIN-5P0: C24.1 C25.+ C27.1 C55.1 C56.1 C59.1 D8.C J6.A4(VBUS) J6.A9(VBUS) J6.B4(VBUS) J6.B9(VBUS) JP2.1 JP3.34 JP4.7 R2.2 R5.2 R62.2 R71.2 R72.2 U2.6(VBUS) U3.1(EN) U3.6(VIN)
VMON_ER_SYS: R1.2 R2.1 U1.A15(B:VMON_ER_SYS)
VOUT0_DATA0: JP2.21 U1.P26(H:VOUT0_DATA0)
VOUT0_DATA1: JP3.21 U1.N25(H:VOUT0_DATA1)
VOUT0_DATA2: JP2.22 U1.N26(H:VOUT0_DATA2)
VOUT0_DATA3: JP3.22 U1.M25(H:VOUT0_DATA3)
VOUT0_DATA4: JP2.23 U1.M26(H:VOUT0_DATA4)
VOUT0_DATA5: JP3.23 U1.U27(H:VOUT0_DATA5)
VOUT0_DATA6: JP2.24 U1.T27(H:VOUT0_DATA6)
VOUT0_DATA7: JP3.24 U1.T28(H:VOUT0_DATA7)
VOUT0_DATA8: JP2.25 U1.R27(H:VOUT0_DATA8)
VOUT0_DATA9: JP3.25 U1.R28(H:VOUT0_DATA9)
VOUT0_DATA10: JP2.26 U1.P27(H:VOUT0_DATA10)
VOUT0_DATA11: JP3.26 U1.P28(H:VOUT0_DATA11)
VOUT0_DATA12: JP2.27 U1.N27(H:VOUT0_DATA12)
VOUT0_DATA13: JP3.27 U1.N28(H:VOUT0_DATA13)
VOUT0_DATA14: JP2.28 U1.M27(H:VOUT0_DATA14)
VOUT0_DATA15: JP3.28 U1.M28(H:VOUT0_DATA15)
VOUT0_DE: JP2.19 U1.R25(H:VOUT0_DE)
VOUT0_HSYNC: JP3.20 U1.P25(H:VOUT0_HSYNC)
VOUT0_PCLK: JP3.19 U1.T26(H:VOUT0_PCLK)
VOUT0_VSYNC: JP2.20 U1.R26(H:VOUT0_VSYNC)
VPP: C62.1 U1.C16(A:VPP) U14.1(OUT)
VPP_EN: J1.2 R3.2 U14.3(EN)
WKUP_CLKOUT0: JP5.15 U1.C7(D:WKUP_CLKOUT0)
WKUP_I2C0_SCL: J4.13 R64.1 U1.A8(D:WKUP_I2C0_SCL)
WKUP_I2C0_SDA: J4.14 R12.1 U1.B8(D:WKUP_I2C0_SDA)
WKUP_LFOSC0_XI: U1.H1(D:WKUP_LFOSC0_XI) Y1.3(OUT)
WKUP_UART0_CTSN: JP5.6 U1.D1(D:WKUP_UART0_CTSN)
WKUP_UART0_RTSN: JP5.7 U1.D2(D:WKUP_UART0_RTSN)
WKUP_UART0_RXD: JP5.9 U1.C2(D:WKUP_UART0_RXD)
WKUP_UART0_TXD: JP5.8 U1.C1(D:WKUP_UART0_TXD)
Unconnected: FUD1.P$1 FUD2.P$1 FUD3.P$1 FUD4.P$1 FUD5.P$1 FUD6.P$1 J4.1_1 J4.2_1 J4.3_1 J4.4_1 J4.5_1 J4.6_1 J4.7_1 J4.8_1 J4.9_1 J4.10_1 J4.11_1 J4.12_1 J4.13_1 J4.14_1 J4.15_1 J5.A8(SBU1) J5.B8(SBU2) J6.A8(SBU1) J6.B8(SBU2) J8.4 J8.5 U1.F4(K:AM62X_RSVD1) U1.F5(K:AM62X_RSVD0) U1.F6(K:AM62X_RSVD2) U1.F7(K:AM62X_RSVD8) U1.F8(K:AM62X_RSVD4) U1.F9(K:AM62X_RSVD5) U1.F10(K:DDR_RSVD0) U1.F15(L:AM62X_DNU11) U1.F16(L:AM62X_DNU12) U1.J2(L:AM62X_DNU13) U1.M14(L:AM62X_DNU10) U1.M18(K:AM62X_RSVD6) U1.M19(L:AM62X_DNU14) U1.N17(K:AM62X_RSVD3) U1.N18(K:AM62X_RSVD7) U1.N19(L:AM62X_DNU15) U1.R15(L:AM62X_DNU9) U1.R16(L:AM62X_DNU8) U1.R17(L:AM62X_DNU7) U1.R18(L:AM62X_DNU6) U1.T15(L:AM62X_DNU5) U1.T16(L:AM62X_DNU4) U1.T17(L:AM62X_DNU3) U1.T18(L:AM62X_DNU2) U1.U13(F:CSI0_RXN3) U1.U14(F:CSI0_RXN2) U1.U18(L:AM62X_DNU1) U1.V13(F:CSI0_RXP3) U1.V14(F:CSI0_RXP2) U1.V18(L:AM62X_DNU0) U2.3(ID) U2.5(N.C.) U3.2(PG) U6.8(GPO1) U6.16(GPIO) U9.3(ID) U9.5(N.C.) U10.4(CT) U11.1(NC) U11.5(NC) Y1.1(NC)

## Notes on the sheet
- IO Headers | OLDI / LVDS Display Interface | Design Notes
- Connectors support two (2) Mikroe Click Interfaces on the inner headers (East / West)
- Based on AM62x SKEVM with Fulton PMIC
- Supports:  SK-LCD1 Interface (https://www.ti.com/tool/SK-LCD1)
- Revision 1A
    - Intial Revision - Pre-Production
  
  Revision 1B
    - Fixed issue with USB connector shorting power and ground
    - Updated SD card connections to fix UHS-I speed transition
    - Updated PC / PD headers
  
  Revision 1C
    - Added inverter on microSD card CD pin
    - Added back current protection for USB-C UFP connector
    - Added LVDS connector
    - Moved all components to top side of the board (except LVDS connector) 
  
  Revision 1D
    - Added buffer for UART
    - Added buffer for LVDS
    - Updated LVDS documentation
    - Added LDO for VPP per AM62x SKEVM
- SOUTH Connector | NORTH Connector | Need a 40 pin FPC cable 0.5mm pitch  (A Type) cable to connect to the screen.
- WEST
- GPIO1_30 | PWM1_A
- 1 | GPIO1_16 | GPIO1_36
- LVDS length requirements:
    - Inter pair:  0.15mm
    - Intra pair:  5mm
- CS0 | CLICK 0
- CLK | UART2
- D0
- SPI2 | D1 | I2C3
- Buffer to prevent back current on INT / RESET
- This Page Intentionally Left Blank
- I2C1 | CLICK 1 | SPI0
- 40 | UART5
- GPIO1_14 | GPIO1_8
- PWM0_A
- EAST
- GPIO1_7
- PA | PB | PC | PD
- Click Modules come with I2C pull ups on-board.  
  Footprints added on I2C1 and I2C3 for convenience (see other page).
- GPMC[0:15] are used as boot mode pins and have default pull up / pull 
  down behavior.  See "Boot Mode" section for more information.
- To meet the Mikroe Click standard, a resistor mux is used to add GPIO
  functionality to the CLICK0_AN and CLICK1_AN pins.  This is generally 
  not needed in a design based on the OSD62-PM-BRK.
- 9/12 | 1D | 10/12 | 1D | 11/12 | 1D | 12/12 | 1D
- SD Power Load switch
- USB-C Back Current Protection
  Allows USB connection when 
  board is externally powered.
  (Max Vf = 400mV @ 2A)
- I2C0 Pull-up Resistors
- Boot Modes Decode:
    1, PLL Config     B[2:0]     = 0b011          : Ref Clock = 25MHz
    2, Primary Boot  B[9:3]     = 0b1001000 : SDCard FS Boot
    3, Backup Boot  B[13:10] = 0b1011        : UART Boot
- OSD62-PM Signals | USB-C Connector | Oscillators | Power Management | Boot Mode | MicroSD
- Test Points for unused control signals. | Only supports USB2.0; Cannot supply power
- See https://www.ti.com/lit/an/slvafd0a/slvafd0a.pdf
    - Using TPS6521903
- OSD62x 25 MHz Oscillator | OSD62x 32 kHz Oscillator
- UFP Request:  3.0A
- 1.8V only | 1.8V only
- I2C Address:  0x30 (7-bit)
- BOOTMODE 0 | 1
- TFM201610ALC-R47MTAA | BOOTMODE 1 | 1
- Note: VDDSHV5 is used for this interface.
  LDO1 from the PMIC supports both 1.8V
  and 3.3V operation to support SD3.0 speed
- BOOTMODE 2 | 0
- BOOTMODE 3 | 0
- Unused | BOOTMODE 4 | 0
- BOOTMODE 5 | 0
- USBx_VBUS is a power sense 
  input to the AM6254 and 
  must be scaled (see AM6254
  datasheet Section 9.2.3)
- BOOTMODE 6 | 1
- Note: The AM62x ROM code requires CD 
  to have an active-low polarity.  Depending 
  on the CD polarity of the SD card holder
  you may need to add an inverter as shown.
- BOOTMODE 7 | 0
- BOOTMODE 8 | 0
- Unused | AOTA-B160808SR47MT | BOOTMODE 9 | 1
- BOOTMODE 10 | 1
- BOOTMODE 11 | 1
- BOOTMODE 12 | 0
- BOOTMODE 13 | 1
- Pull-up Resistors | BOOTMODE 14 | 0
- BOOTMODE 15 | 0
- CSI Connector | LEDs | Power Button
- Compatible with Raspberry Pi camera connector
- AM62 JTAG Resistors
- ADCs | JTAG Headers
- CSI length requirements:
    - Inter pair:  0.15mm
    - Intra pair:  1.5mm
- For Click Connectors
- Tag Connect
- GPIO1_50
- GPIO1_51
- Oscillator used 
  instead of Crystal
- AM62 Reset Resistors
- USR2 | USR3 | USR1 | USR0
- I2C Addr:  0x51 | I2C Addr:  0x52
- GPIO1_49
- 3.3V DC-DC Converter | I2C Pull Ups
- These are not necessary for designs that do not use the I2C busses.
- Main 3.3V Input
- No pull ups for the Click I2C Interfaces, per spec.
  Footprints added for conveniece.
- TFM201610ALC-R47MTAA
- PMIC_VSEL_SD requires an external pull up to the voltage of the IO bank that drives it.
  This is VDDSHV0, i.e. VIN-3P3-LS, (MMC1_SDWP) for this design.
- EEPROM | USB Connector | UART Header
- Vertical USB Host Port (Type-C) | Buffer added to prevent back current
- Oscillator used 
  instead of Crystal
- USBx_VBUS is a power sense 
  input to the AM6254 and 
  must be scaled (see AM6254
  datasheet Section 9.2.3)
- Click 0
- Click 1
- 4A DC-DC converter | 6A Load Switch
- DFP Advertisement:  
      Default USB Power (500mA/900mA)
- 5/12 | 1D | 6/12 | 1D | 7/12 | 1D | 8/12 | 1D
- 0201 | 0402
- Table of Contents | Power Block Diagram | OSD62-PM Power
- Octavo Systems OSD62-PM-BRK
  
  (c) Copyright, Octavo Systems LLC, 2024-2025. All Rights Reserved.
- 0.01uF | 0.1uF | 1uF | 2.2uF | 4.7uF | 10uF | OSD62-PM Ground | OSD62-PM I/O Power
- Sheet 1:  Title
- All IO to headers on OSD62-PM are 3.3V.
  
  Other designs will need to set VDDSHV banks to meet their IO voltage needs.
- VDD_CORE | 0/3 | 1/0 | 1/0 | 0/1
- TLV62595 | TPS6521903 | OSD62-PM
- Sheet 2:  Notes / Block Diagram / Mechanical
- 3.3V | 0.75V | 0.75V @ 3.5A
- Buck 1 
  0.75V @ 2850mA
- VDDA_CORE_CSIRX0 | 1/0 | 0/1 | 0/0
- 5.0V USB-C
  External Input
- VIN-B1/2/3 | Buck 1 | VDD_CORE | VDDA_CORE_CSIRX0
- Sheet 3:  OSD62-PM Power | VDD_CANUART | VDDA_CORE_USB
- Buck 1
  (0.75 V)
- VDDA_DDR_PLL0 | VDDA_CORE_USB | 1/0 | 0/1
- USB-C
  UFP
- DC-DC 4A
  5.0V to 3.3V
- 1.8V @ 2A
- Buck 2 
  1.8V @ 400mA
- 20mA
- Sheet 4:  OSD62-PM GND / IO Power
- USB-C Back
  Current Protection
- VIN-LDO1 | Buck 2
- TLV75518P
  LDO
- VPP
- VIN-LDO34 | 20mA | VDD_CANUART | 1/0 | 0/1
- THERE IS NO WARRANTY FOR THIS DESIGN, TO THE EXTENT PERMITTED BY APPLICABLE 
  LAW. EXCEPT WHEN OTHERWISE STATED IN WRITING THE COPYRIGHT HOLDERS AND/OR 
  OTHER PARTIES PROVIDE THE DESIGN *AS IS* WITHOUT WARRANTY OF ANY KIND, 
  EITHER EXPRESSED OR IMPLIED, INCLUDING, BUT NOT LIMITED TO, THE IMPLIED 
  WARRANTIES OF MERCHANTABILITY AND FITNESS A FOR A PARTICULAR PURPOSE. 
  THE ENTIRE RISK AS TO THE QUALITY AND PERFORMANCE OF THE DESIGN IS WITH YOU. 
  SHOULD THE DESIGN PROVE DEFECTIVE, YOU ASSUME THE COST OF ALL NECESSARY 
  SERVICING, REPAIR OR CORRECTION.
- 10mA
- Sheet 5:  OSD62-PM Signals | 1.2V @ 2A
- Buck 3 
  1.2V @ 600mA
- 20mA
- Buck 3 | VDDS_DDR
- VDDS_DDR 
  (includes DDR4 VDD/VDDQ)
- 20mA | 1/3 | 1/0 | 1/0 | 1/0 | 30mA
- Sheet 6:  USB-C / CSI / Power In / Osc
- Buck 3
  (1.2 V)
- 1.8V / 3.3V @ 400mA
- LDO 1
  1.8V/3.3V @ 80mA
- 20mA | VDDS_DDR_C
- LDO 1 | VDDSHV5 (microSD) | 30mA
- Sheet 7:  Power Management | Total Core:  3100mA | 20mA
- USB-C
  DFP
  
  500mA
- Buck 2 Input
    - Required due to 
      power sequencing
- VDDR_CORE | 0/3 | 1/0 | 1/0
- 0.85V @ 400mA
- LDO 2 
  0.85V @ 80mA
- VDDR_CORE | 30mA
- LDO2
  (0.85 V)
- 30mA
- Sheet 8:  JTAG / Boot Mode / microSD / etc. | VIN-LDO2 | LDO 2 | VDDS_DDR_C
- VDDA_1P8_OLDI0 | 1/0 | 0/1 | 0/1
- 30mA
- Sheet 9:  IO Headers | 1.8V @ 300mA
- LDO 3 
  1.8V @ 200mA
- VDDS_OSC0 | VDDA_1P8_CSIRX0
- LDO 3 | VDDA_MCU | VDDA_1P8_OLDI0
- LDO3
  (1.8 V)
- VDDA_1P8_CSIRX0 | 1/0 | 0/1 | 0/1
- VDDA_PLLx | VDDA_1P8_USB | 5mA | 30mA
- Sheet 10:  LVDS Connector | VDDA_TEMPx | 40mA
- 2.5V @ 300mA
- LDO 4 
  2.5V @ 60mA
- VDDA_1V8_USB | 1/0 | 0/1
- GPO2 | LDO 4 | DDR_VPP | 30mA
- Sheet 11:  Blank | 400mA
- VDDA_1V8_MCU | 1/0
- 30mA
- Sheet 12:  Design Notes | 10mA | 50mA
- TPS22965 | VDDA_1V8_PLL0 | 1/0
- 30mA
- 3.3V
- EN | VDDA_3P3_USB | 250mA | 200mA | VDDA_1V8_PLL1 | 1/0
- Load Switch
  6A
- VDDA_1V8_PLL2 | 1/0
- OSD62-PM BRK | VDDSHV_CANUART
- VDDSHV_MCU
- VDDSHV0 | Internal PM / OSD62 BRK Board
- VDDSHV1
- VDDSHV2
- See Documents:  
    - https://www.ti.com/lit/an/sprac76f/sprac76f.pdf  (see page 29)
    - https://www.ti.com/lit/zip/spar001 (See Sheet 14)
- To
  System
- VDDSHV3 | 200mA
- VDDSHV4
- VDDSHV6
- USB-C Power Discussion
- Maximum Current Requirements:
    - https://www.ti.com/lit/an/sprada6/sprada6.pdf
- The USB-C UFP uses 5.1k pull down resistors on the CC pins to request up to 3A from the DFP.  However, this board does not check the voltage of the CC pins to understand the current provided by the DFP port.  The USB-C DFP port 
  on this board uses 56k ohm pull up resistors to advertise 500mA of current availlable.  It is the resposibility of the user to guarantee that there is enough current to support both the components on the board as welll as any downstream
  USB devices.
- Version 1D
- VPP LDO
- I2C Table | Mechanical & Misc | OSD62-PM Reserved / DNU
- I2C0 | Fiducials
- ADDRESS | DEVICE
- 0x13 | TPS65219
- 0x50 | EEPROM
- 0x51 | ADC121C027
- 0x52 | ADC121C027
- 1/12 | 1D | 2/12 | 1D | 3/12 | 1D | 4/12 | 1D

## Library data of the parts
C1-C3 C6-C15 C17-C20 C61 = OSD62-PM-BRK:C: Capacitor SMD.; SIZE: 0201; VOLTAGE: 6.3V
C4 C24 C26 C29 C34-C36 C46 C50 C54 C55 C58 C59 C62 C63 = OSD62-PM-BRK:C: Capacitor SMD.; SIZE: 0402; VOLTAGE: 6.3V
C5 C16 C21-C23 C30 C38-C45 C48 C51 C52 C60 = OSD62-PM-BRK:C: Capacitor SMD.; SIZE: 0402; VOLTAGE: 10V
C25 = OSD62-PM-BRK:CPOL-US: POLARIZED CAPACITOR, American symbol
C27 C31-C33 C37 C57 = OSD62-PM-BRK:C: Capacitor SMD.; SIZE: 0603; VOLTAGE: 10V
C28 = OSD62-PM-BRK:C: Capacitor SMD.; SIZE: 0402
C47 C49 C53 = OSD62-PM-BRK:C: Capacitor SMD.; SIZE: 0603; VOLTAGE: 6.3V
C56 = OSD62-PM-BRK:C: Capacitor SMD.; SIZE: 0805; VOLTAGE: 10V
D1-D5 = OSD62-PM-BRK:LTST-C191TBKT: PointLED® Enhanced Thinfilm LED TOP & BOTTOM mount
D6 D7 = OSD62-PM-BRK:RB520S30T1G
D8 = OSD62-PM-BRK:RBS2MM40C: Schottky Diode: 2A, 40V - Footprint also supports: SD1206S040L2R0
FUD1-FUD6 = OSD62-PM-BRK:FIDUCIAL
J1 J2 J7 = OSD62-PM-BRK:PINHD-1X2: 2-pin 100 mil header
J4 = OSD62-PM-BRK:1-1734248-5: CONN FPC VERT 15POS 1.00MM SMD Check availability; AVAILABILITY: In Stock; CHECK_PRICES: https://www.snapeda.com/parts/1-1734248-5/TE+Connectivity+AMP+Connectors/view-part/?ref=eda; COMMENT: 1-1734248-5; DESCRIPTION: 15 Position FPC Connector Contacts, Vertical - 1 Sided 0.039 (1.00mm) Surface Mount; MF: TE Connectivity; MP: 1-1734248-5; PACKAGE: None; PRICE: None; PURCHASE-URL: https://www.snapeda.com/api/url_track_click_mouser/?unipart_id=618488&manufacturer=TE Connectivity&part_name=1-1734248-5&search_term=1-1734248-5; SNAPEDA_LINK: https://www.snapeda.com/parts/1-1734248-5/TE+Connectivity+AMP+Connectors/view-part/?ref=snap
J5 = OSD62-PM-BRK:USB4105-GF-A: Check availability; AVAILABILITY: In Stock; CHECK_PRICES: https://www.snapeda.com/parts/USB4105-GF-A/Global+Connector+Technology/view-part/?ref=eda; DESCRIPTION: USB-C (USB TYPE-C) USB 2.0 Receptacle Connector 24 (16+8 Dummy) Position Surface Mount, Right Angle; Through Hole; MF: GCT; MP: USB4105-GF-A; PACKAGE: None; PRICE: None; PURCHASE-URL: https://www.snapeda.com/api/url_track_click_mouser/?unipart_id=4423780&manufacturer=GCT&part_name=USB4105-GF-A&search_term=usb4105-gf-a; SNAPEDA_LINK: https://www.snapeda.com/parts/USB4105-GF-A/Global+Connector+Technology/view-part/?ref=snap
J6 = OSD62-PM-BRK:2171820001: Check availability; AVAILABILITY: In Stock; CHECK_PRICES: https://www.snapeda.com/parts/217182-0001/Molex/view-part/?ref=eda; DESCRIPTION: USB Type C - Connector, Vertical SMT L6.4 16pos | Molex Incorporated 217182-0001; MF: Molex; MP: 217182-0001; PACKAGE: None; PRICE: None; PURCHASE-URL: https://www.snapeda.com/api/url_track_click_mouser/?unipart_id=6306497&manufacturer=Molex&part_name=217182-0001&search_term=2171820001; SNAPEDA_LINK: https://www.snapeda.com/parts/217182-0001/Molex/view-part/?ref=snap
J8 = OSD62-PM-BRK:505110-4091: 40 Position FFC, FPC Connector Contacts, Bottom 0.020" (0.50mm) Surface Mount, Right Angle Check availability; AVAILABILITY: In Stock; DESCRIPTION: 40 Position FFC, FPC Connector Contacts, Bottom 0.020 (0.50mm) Surface Mount, Right Angle; MF: Molex; MP: 5051104091; PACKAGE: None; PRICE: None; PURCHASE-URL: https://pricing.snapeda.com/search/part/5051104091/?ref=eda
JP1 = OSD62-PM-BRK:PINHD-1X3: PIN HEADER
JP2-JP5 = OSD62-PM-BRK:PINHD-1X40: PIN HEADER
L1 L4 = OSD62-PM-BRK:L; CURRENT: 5.2A; SIZE: 0806
L2 L3 = OSD62-PM-BRK:L; CURRENT: 3A; SIZE: 0603
R1-R5 R7 R10-R34 R37-R74 R76 = OSD62-PM-BRK:R-US_: RESISTOR, American symbol; SIZE: 0402; TOLERANCE: 5%
R6 R8 R9 R35 R36 = OSD62-PM-BRK:R-US_: RESISTOR, American symbol; SIZE: 0402; TOLERANCE: 1%
S1 = OSD62-PM-BRK:TACT: Library: MF_Switches Description: Device for Tact Switches. Manufacture part number (MFG#) can be added via Attributes.; HOUSEPART: YES; MPN: MF-SW-TACT-4.2MM; POPULATE: 1; URL: https://factory.macrofab.com/part/MF-SW-TACT-4.2MM
TC1 = OSD62-PM-BRK:TC2050-IDC: Tag-Connect In Circuit Programming & Debug Cable 10 Pin http://www.tag-connect.com
TP1-TP3 TP6 TP7 = OSD62-PM-BRK:TP: Test pad
U1 = OSD62-PM-BRK:OSD6254-1G-BPM-ES: OSD62x-SO BGA Array
U2 U9 = OSD62-PM-BRK:TPD4S012_DRY_6
U3 = OSD62-PM-BRK:TLV62595DMQR
U4 = OSD62-PM-BRK:24AA32A
U5 = OSD62-PM-BRK:TPS22965DSGT: 5.7-V, 6-A, 16-mΩ load switch with adj. rise time and optional output discharge Check availability; AVAILABILITY: In Stock; CHECK_PRICES: https://www.snapeda.com/parts/TPS22965DSGT/Texas+Instruments/view-part/?ref=eda; DESCRIPTION: 5.7-V, 6-A, 16-mΩ load switch with adj. rise time and optional output discharge; MF: Texas Instruments; MP: TPS22965DSGT; PACKAGE: WSON-8 Texas Instruments; PRICE: None; PURCHASE-URL: https://www.snapeda.com/api/url_track_click_mouser/?unipart_id=208538&manufacturer=Texas Instruments&part_name=TPS22965DSGT&search_term=tps22965dsgt; SNAPEDA_LINK: https://www.snapeda.com/parts/TPS22965DSGT/Texas+Instruments/view-part/?ref=snap
U6 = OSD62-PM-BRK:TPS65219
U7 U8 = OSD62-PM-BRK:ADC121C027CIMK: Check availability; AVAILABILITY: In Stock; DESCRIPTION: I2C-Compatible, 12-Bit Analog-to-Digital Converter with Alert Function 6-SOT-23-THIN -40 to 105; MF: Texas Instruments; MP: ADC121C027CIMK/NOPB; PACKAGE: SOT-23-THN-6 Texas Instruments; PRICE: None; PURCHASE-URL: https://pricing.snapeda.com/search/part/ADC121C027CIMK/NOPB/?ref=eda
U10 = OSD62-PM-BRK:TPS22918DBVR: Check availability; AVAILABILITY: In Stock; CHECK_PRICES: https://www.snapeda.com/parts/TPS22918DBVR/Texas+Instruments/view-part/?ref=eda; DESCRIPTION: 5.5-V, 2-A, 52-mΩ load switch with adj. rise time and adj. output discharge; MF: Texas Instruments; MP: TPS22918DBVR; PACKAGE: SOT-23-6 Texas Instruments; PRICE: None; PURCHASE-URL: https://www.snapeda.com/api/url_track_click_mouser/?unipart_id=490084&manufacturer=Texas Instruments&part_name=TPS22918DBVR&search_term=tps22918dbvr; SNAPEDA_LINK: https://www.snapeda.com/parts/TPS22918DBVR/Texas+Instruments/view-part/?ref=snap
U11 = OSD62-PM-BRK:SN74LVC1G04DSFR: Check availability; AVAILABILITY: In Stock; CHECK_PRICES: https://www.snapeda.com/parts/SN74LVC1G04DSFR/Texas+Instruments/view-part/?ref=eda; DESCRIPTION: Single 1.65-V to 5.5-V inverter; MF: Texas Instruments; MP: SN74LVC1G04DSFR; PACKAGE: X2SON-6 Texas Instruments; PRICE: None; SNAPEDA_LINK: https://www.snapeda.com/parts/SN74LVC1G04DSFR/Texas+Instruments/view-part/?ref=snap
U12 U13 = OSD62-PM-BRK:SN74LVC2G241YZPR
U14 = OSD62-PM-BRK:TLV75518P
X1 = OSD62-PM-BRK:SD_CARD_SLOT: Library: MF_Connectors Description: SD Card Connector; HOUSEPART: YES; MPN: MF-MICROSD; POPULATE: 1; URL: https://factory.macrofab.com/part/MF-MICROSD
Y1 = OSD62-PM-BRK:SIT1533AI-H4-D14-32.768
Y2 = OSD62-PM-BRK:SIT8008BI-73-YYS-25.000000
